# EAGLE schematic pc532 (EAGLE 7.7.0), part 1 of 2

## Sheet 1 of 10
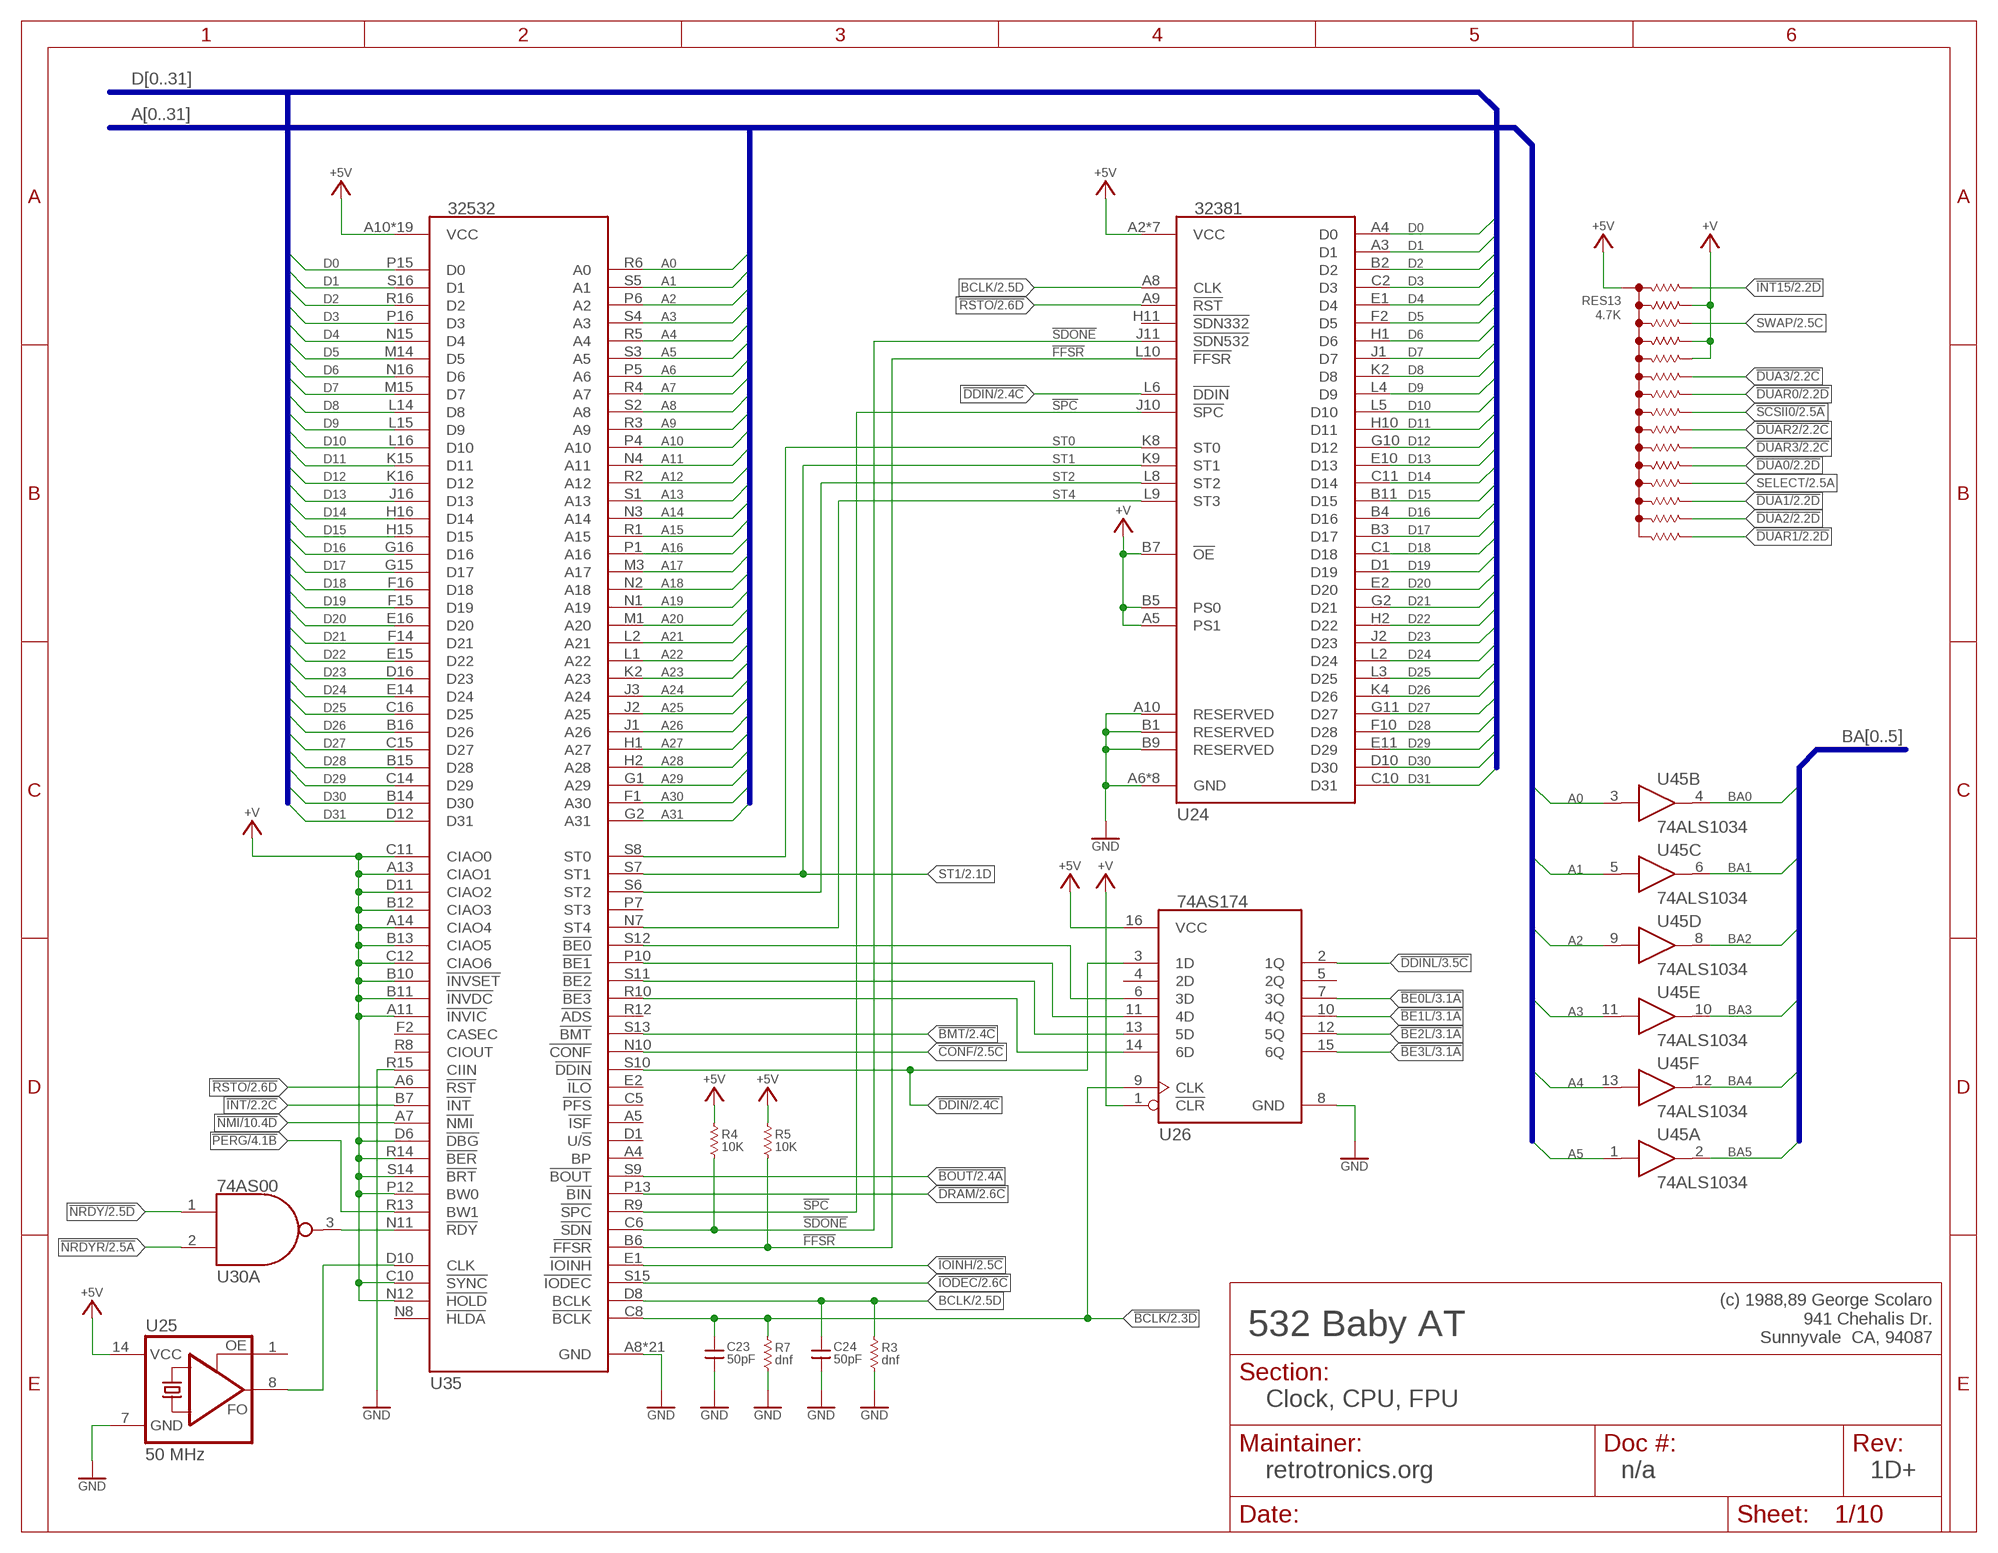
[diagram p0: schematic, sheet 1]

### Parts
C23  50pF  C_US_300M  [C_TH_300MIL]
C24  50pF  C_US_300M  [C_TH_300MIL]
R3  dnf  R_US  [R_204/7]
R4  10K  R_US  [R_204/7]
R5  10K  R_US  [R_204/7]
R7  dnf  R_US  [R_204/7]
RES13  4.7K  RNET_X15  [DIL16]
U24  32381  [PGA68]
U25  50 MHz  XTAL_CAN_HALFSIZEFP  [DIL14]
U26  74AS174  74174  [DIL16]
U30  74AS00  7400  [DIL14]
U35  32532  [PGA175]
U45  74ALS1034  7407D  [DIL14]

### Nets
!BCLK: C23.1 R7.2 U26.9(CLK) U35.C8(!BCLK) ; also sheet 2,3
!BE0: U26.6(3D) U35.S12(!BE0)
!BE0L: U26.7(3Q) ; also sheet 3,10
!BE1: U26.11(4D) U35.P10(!BE1)
!BE1L: U26.10(4Q) ; also sheet 3,10
!BE2: U26.13(5D) U35.S11(!BE2)
!BE2L: U26.12(5Q) ; also sheet 3,10
!BE3: U26.14(6D) U35.R10(!BE3)
!BE3L: U26.15(6Q) ; also sheet 3,10
!BMT: U35.S13(!BMT) ; also sheet 2,3
!BOUT: U35.S9(!BOUT) ; also sheet 2
!CONF: U35.N10(!CONF) ; also sheet 2,3
!DDIN: U24.L6(!DDIN) U26.3(1D) U35.S10(!DDIN) ; also sheet 2,3
!DDINL: U26.2(1Q) ; also sheet 3,4
!DRAM: U35.P13(!BIN) ; also sheet 2,3
!DUA0: RES13.11(R11) ; also sheet 2,7
!DUA1: RES13.13(R13) ; also sheet 2,6
!DUA2: RES13.14(R14) ; also sheet 2,7
!DUA3: RES13.6(R6) ; also sheet 2,6
!DUAR0: RES13.7(R7) ; also sheet 2,7
!DUAR1: RES13.15(R15) ; also sheet 2,6
!DUAR2: RES13.9(R9) ; also sheet 2,7
!DUAR3: RES13.10(R10) ; also sheet 2,6
!FFSR: R5.1 U24.L10(!FFSR) U35.B6(!FFSR)
!INT: U35.B7(!INT) ; also sheet 2
!INT15: RES13.1(R1) ; also sheet 2
!IODEC: U35.S15(!IODEC) ; also sheet 2
!IOINH: U35.E1(!IOINH) ; also sheet 2
!NMI: U35.A7(!NMI) ; also sheet 10
!NRDY: U30.1(A:A) ; also sheet 2
!NRDYR: U30.2(A:B) ; also sheet 2
!PERG: U35.R13(BW1) ; also sheet 4
!RDY: U30.3(A:Y) U35.N11(!RDY)
!RSTO: U24.A9(!RST) U35.A6(!RST) ; also sheet 2,4,5,10
!SCSII0: RES13.8(R8) ; also sheet 2,4
!SDONE: R4.1 U24.J11(!SDN532) U35.C6(!SDN)
!SPC: U24.J10(!SPC) U35.R9(!SPC)
+5V: R4.2 R5.2 RES13.16(C) U24.A2(VCC) U24.B10(VCC) U24.D2(VCC) U24.D11(VCC) U24.K1(VCC) U24.K6(VCC) U24.L7(VCC) U25.14(VCC) U26.16(VCC) U35.A10(VCC) U35.A15(VCC) U35.B2(VCC) U35.B5(VCC) U35.B8(VCC) U35.C3(VCC) U35.C9(VCC) U35.C13(VCC) U35.D15(VCC) U35.G3(VCC) U35.H14(VCC) U35.J15(VCC) U35.K1(VCC) U35.L3(VCC) U35.M16(VCC) U35.N13(VCC) U35.P2(VCC) U35.P9(VCC) U35.R11(VCC) ; also sheet 2,3,4,5,6,7,8,9,10
+V: RES13.2(R2) RES13.4(R4) RES13.5(R5) U24.A5(PS1) U24.B5(PS0) U24.B7(!OE) U26.1(!CLR) U35.A11(!INVIC) U35.A13(CIAO1) U35.A14(CIAO4) U35.B10(!INVSET) U35.B11(!INVDC) U35.B12(CIAO3) U35.B13(CIAO5) U35.C10(!SYNC) U35.C11(CIAO0) U35.C12(CIAO6) U35.D6(!DBG) U35.D11(CIAO2) U35.N12(!HOLD) U35.P12(BW0) U35.R14(!BER) U35.S14(!BRT) ; also sheet 2,3,4
A0: U35.R6(A0) U45.3(B:A) ; also sheet 2
A1: U35.S5(A1) U45.5(C:A) ; also sheet 2
A2: U35.P6(A2) U45.9(D:A) ; also sheet 2,3
A3: U35.S4(A3) U45.11(E:A) ; also sheet 2,3
A4: U35.R5(A4) U45.13(F:A) ; also sheet 2,3
A5: U35.S3(A5) U45.1(A:A) ; also sheet 2,3
A6: U35.P5(A6) ; also sheet 2,3
A7: U35.R4(A7) ; also sheet 2,3
A8: U35.S2(A8) ; also sheet 2,3
A9: U35.R3(A9) ; also sheet 2,3
A10: U35.P4(A10) ; also sheet 2,3
A11: U35.N4(A11) ; also sheet 2,3
A12: U35.R2(A12) ; also sheet 2,3
A13: U35.S1(A13) ; also sheet 2,3
A14: U35.N3(A14) ; also sheet 2,3
A15: U35.R1(A15) ; also sheet 2,3
A16: U35.P1(A16) ; also sheet 2,3
A17: U35.M3(A17) ; also sheet 2,3
A18: U35.N2(A18) ; also sheet 2,3
A19: U35.N1(A19) ; also sheet 2,3
A20: U35.M1(A20) ; also sheet 2,3
A21: U35.L2(A21) ; also sheet 2,3
A22: U35.L1(A22) ; also sheet 2,3
A23: U35.K2(A23) ; also sheet 3
A24: U35.J3(A24) ; also sheet 2,3
A25: U35.J2(A25)
A26: U35.J1(A26)
A27: U35.H1(A27) ; also sheet 2
A28: U35.H2(A28) ; also sheet 2
A29: U35.G1(A29) ; also sheet 2
A30: U35.F1(A30) ; also sheet 2
A31: U35.G2(A31) ; also sheet 2
BA0: U45.4(B:Y) ; also sheet 2,4,5,6,7
BA1: U45.6(C:Y) ; also sheet 2,5,6,7
BA2: U45.8(D:Y) ; also sheet 2,5,6,7
BA3: U45.10(E:Y) ; also sheet 2,6,7
BA4: U45.12(F:Y) ; also sheet 2
BA5: U45.2(A:Y) ; also sheet 2
BCLK: C24.1 R3.2 U24.A8(CLK) U35.D8(BCLK) ; also sheet 2,10
CLK: U25.8(FO) U35.D10(CLK)
D0: U24.A4(D0) U35.P15(D0) ; also sheet 4,8,10
D1: U24.A3(D1) U35.S16(D1) ; also sheet 4,8,10
D2: U24.B2(D2) U35.R16(D2) ; also sheet 4,8,10
D3: U24.C2(D3) U35.P16(D3) ; also sheet 4,8,10
D4: U24.E1(D4) U35.N15(D4) ; also sheet 4,8,10
D5: U24.F2(D5) U35.M14(D5) ; also sheet 4,8,10
D6: U24.H1(D6) U35.N16(D6) ; also sheet 4,8,10
D7: U24.J1(D7) U35.M15(D7) ; also sheet 4,8,10
D8: U24.K2(D8) U35.L14(D8) ; also sheet 8,10
D9: U24.L4(D9) U35.L15(D9) ; also sheet 8,10
D10: U24.L5(D10) U35.L16(D10) ; also sheet 8,10
D11: U24.H10(D11) U35.K15(D11) ; also sheet 8,10
D12: U24.G10(D12) U35.K16(D12) ; also sheet 8,10
D13: U24.E10(D13) U35.J16(D13) ; also sheet 8,10
D14: U24.C11(D14) U35.H16(D14) ; also sheet 8,10
D15: U24.B11(D15) U35.H15(D15) ; also sheet 8,10
D16: U24.B4(D16) U35.G16(D16) ; also sheet 8,10
D17: U24.B3(D17) U35.G15(D17) ; also sheet 8,10
D18: U24.C1(D18) U35.F16(D18) ; also sheet 8,10
D19: U24.D1(D19) U35.F15(D19) ; also sheet 8,10
D20: U24.E2(D20) U35.E16(D20) ; also sheet 8,10
D21: U24.G2(D21) U35.F14(D21) ; also sheet 8,10
D22: U24.H2(D22) U35.E15(D22) ; also sheet 8,10
D23: U24.J2(D23) U35.D16(D23) ; also sheet 8,10
D24: U24.L2(D24) U35.E14(D24) ; also sheet 8,10
D25: U24.L3(D25) U35.C16(D25) ; also sheet 8,10
D26: U24.K4(D26) U35.B16(D26) ; also sheet 8,10
D27: U24.G11(D27) U35.C15(D27) ; also sheet 8,10
D28: U24.F10(D28) U35.B15(D28) ; also sheet 8,10
D29: U24.E11(D29) U35.C14(D29) ; also sheet 8,10
D30: U24.D10(D30) U35.B14(D30) ; also sheet 8,10
D31: U24.C10(D31) U35.D12(D31) ; also sheet 8,10
GND: C23.2 C24.2 R3.1 R7.1 U24.A6(GND) U24.A7(GND) U24.A10(RESERVED) U24.B1(RESERVED) U24.B6(GND) U24.B9(RESERVED) U24.F11(GND) U24.G1(GND) U24.K3(GND) U24.K5(GND) U24.K11(GND) U25.7(GND) U26.8(GND) U35.A8(GND) U35.A12(GND) U35.B9(GND) U35.D4(GND) U35.D5(GND) U35.D9(GND) U35.D13(GND) U35.D14(GND) U35.E3(GND) U35.G14(GND) U35.H3(GND) U35.J14(GND) U35.K3(GND) U35.K14(GND) U35.M2(GND) U35.N6(GND) U35.N9(GND) U35.N14(GND) U35.P3(GND) U35.P8(GND) U35.P11(GND) U35.R15(CIIN) ; also sheet 2,3,4,5,6,7,8,9,10
SELECT: RES13.12(R12) ; also sheet 2
ST0: U24.K8(ST0) U35.S8(ST0)
ST1: U24.K9(ST1) U35.S7(ST1) ; also sheet 2
ST2: U24.L8(ST2) U35.S6(ST2)
ST4: U24.L9(ST3) U35.N7(ST4)
SWAP: RES13.3(R3) ; also sheet 2
Unconnected: U24.H11(!SDN332) U25.1(OE) U26.4(2D) U26.5(2Q) U35.A4(BP) U35.A5(!ISF) U35.C5(!PFS) U35.D1(U/!S) U35.E2(!ILO) U35.F2(CASEC) U35.N8(!HLDA) U35.P7(ST3) U35.R8(CIOUT) U35.R12(!ADS)

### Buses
D[0..31]
A[0..31]
BA[0..5]

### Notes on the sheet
- (c) 1988,89 George Scolaro
  941 Chehalis Dr.
  Sunnyvale  CA, 94087
- 532 Baby AT
- Clock, CPU, FPU
- retrotronics.org | n/a | 1D+

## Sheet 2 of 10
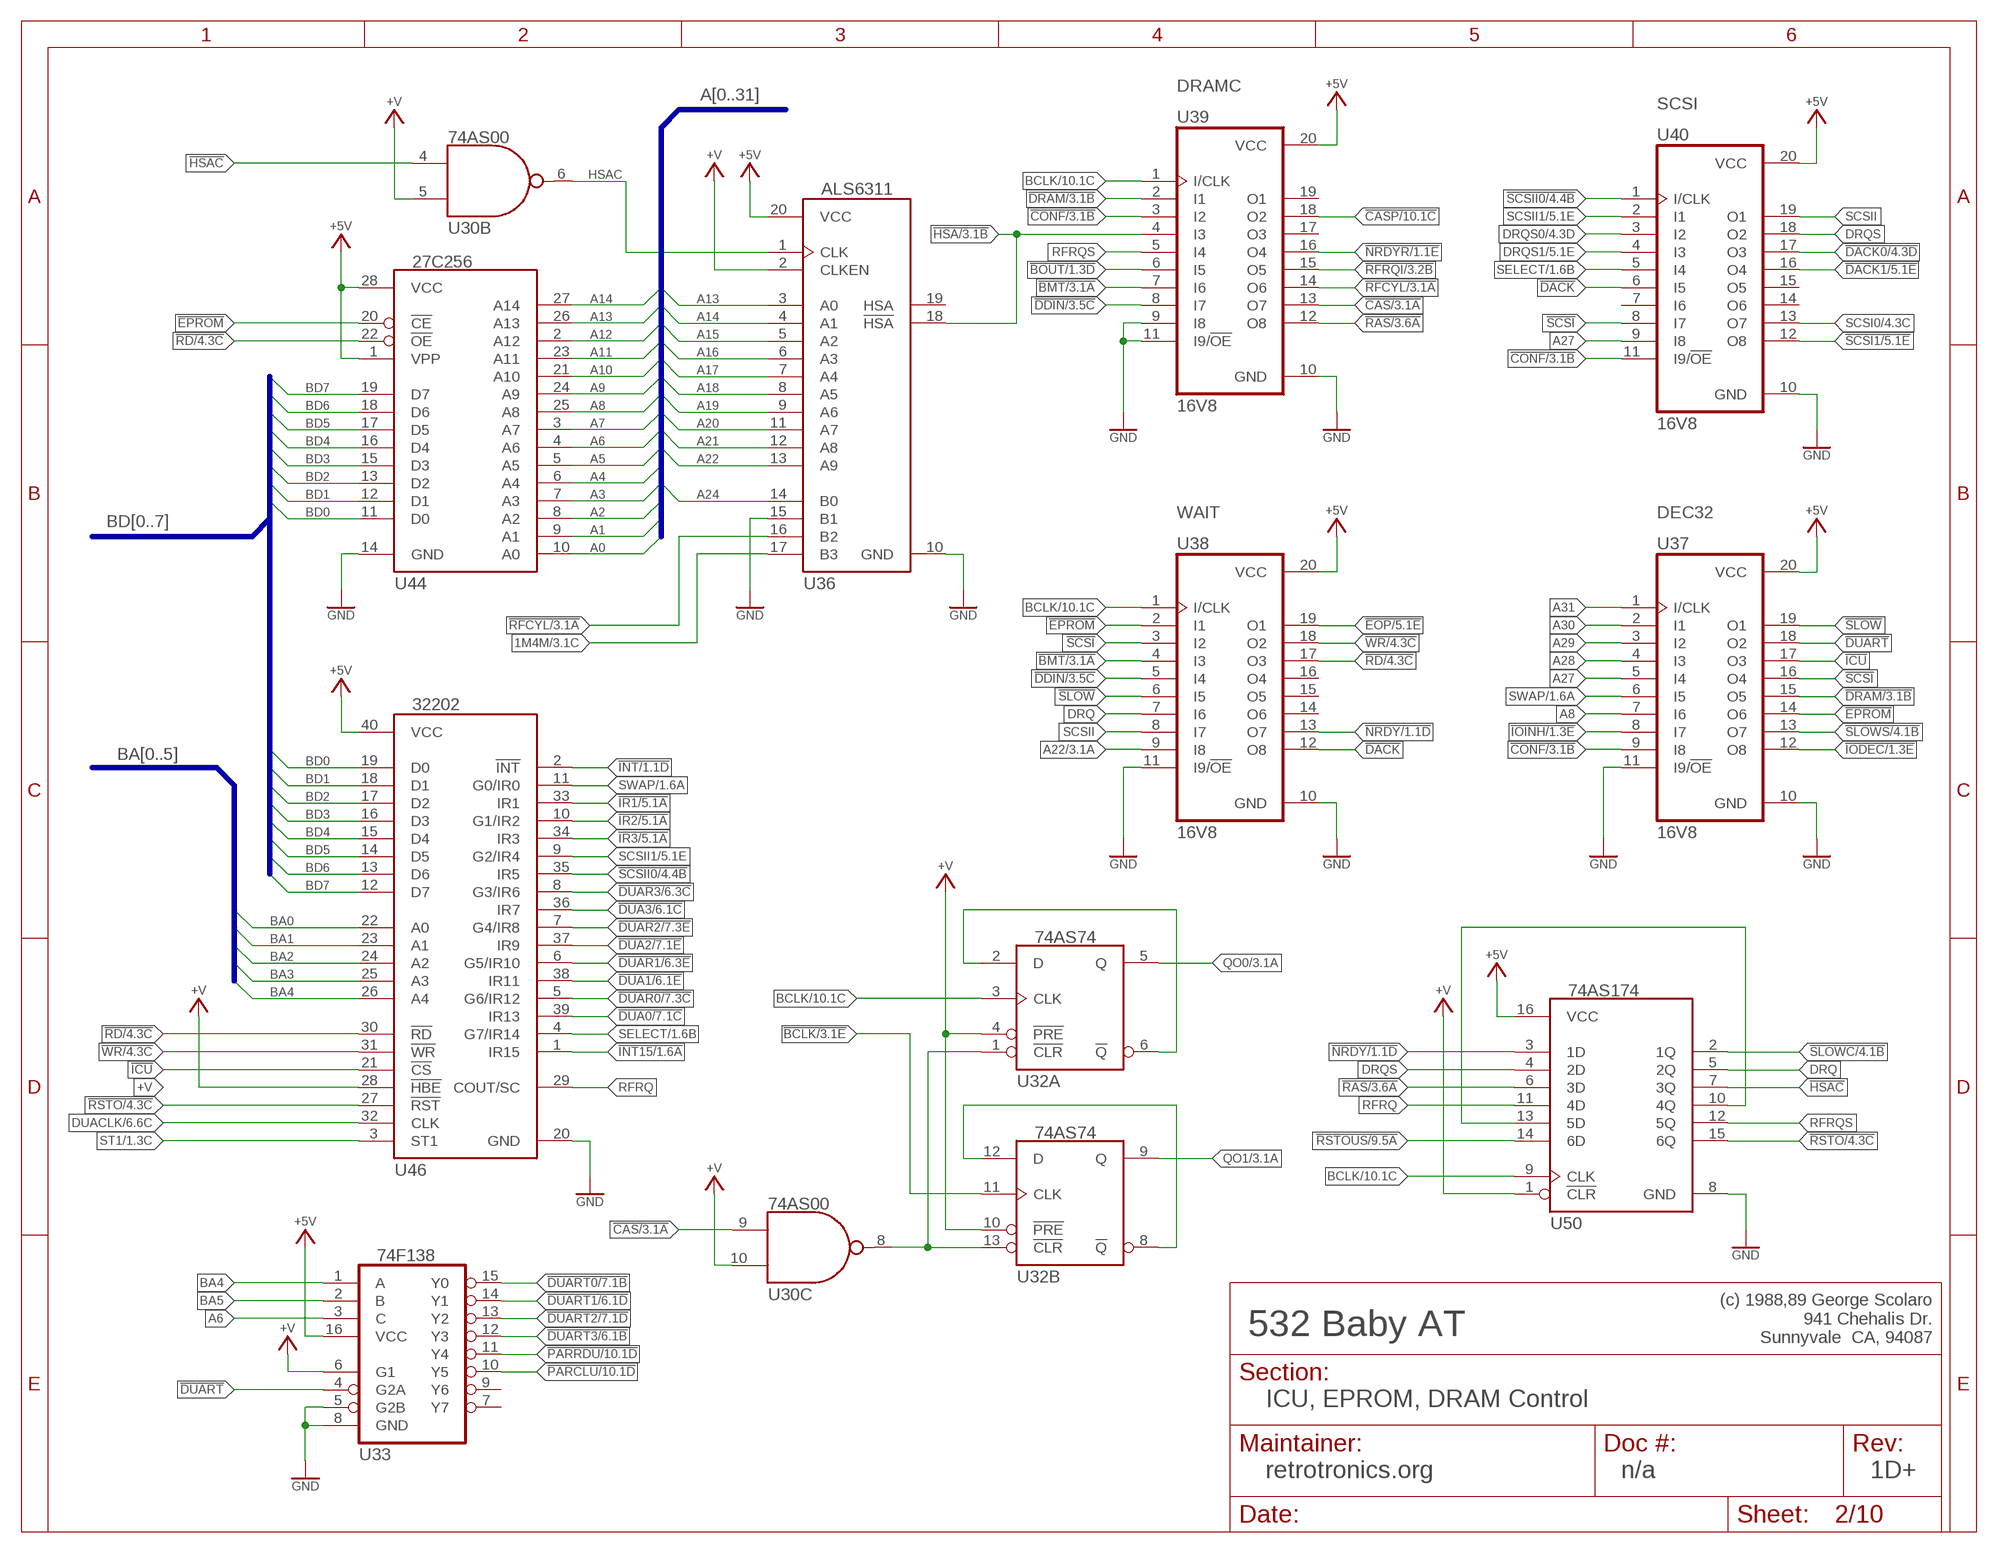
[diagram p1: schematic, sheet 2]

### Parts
U32  74AS74  7474  [DIL14]
U33  74F138  74138  [DIL16]
U36  ALS6311  746311  [DIL20]
U37  16V8  16V8_RND  [DIL20_ROUND]
U38  16V8  16V8_RND  [DIL20_ROUND]
U39  16V8  16V8_RND  [DIL20_ROUND]
U40  16V8  16V8_RND  [DIL20_ROUND]
U44  27C256  [DIL28W]
U46  32202  [DIL40]
U50  74AS174  74174  [DIL16]

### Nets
1M4M: U36.17(B3) ; also sheet 3
!BCLK: U32.11(B:CLK) ; also sheet 1,3
!BCLK_CLR: U30.8(C:Y) U32.1(A:!CLR) U32.13(B:!CLR)
!BMT: U38.4(I3) U39.7(I6) ; also sheet 1,3
!BOUT: U39.6(I5) ; also sheet 1
!CAS: U30.9(C:A) U39.13(O7) ; also sheet 3
!CASP: U39.18(O2) ; also sheet 10
!CONF: U37.9(I8) U39.3(I2) U40.11(I9/!OE) ; also sheet 1,3
!DACK: U38.12(O8) U40.6(I5)
!DACK0: U40.17(O3) ; also sheet 4
!DACK1: U40.16(O4) ; also sheet 5
!DDIN: U38.5(I4) U39.8(I7) ; also sheet 1,3
!DRAM: U37.15(O5) U39.2(I1) ; also sheet 1,3
!DUA0: U46.39(IR13) ; also sheet 1,7
!DUA1: U46.38(IR11) ; also sheet 1,6
!DUA2: U46.37(IR9) ; also sheet 1,7
!DUA3: U46.36(IR7) ; also sheet 1,6
!DUAR0: U46.5(G6/IR12) ; also sheet 1,7
!DUAR1: U46.6(G5/IR10) ; also sheet 1,6
!DUAR2: U46.7(G4/IR8) ; also sheet 1,7
!DUAR3: U46.8(G3/IR6) ; also sheet 1,6
!DUART: U33.4(G2A) U37.18(O2)
!DUART0: U33.15(Y0) ; also sheet 7
!DUART1: U33.14(Y1) ; also sheet 6
!DUART2: U33.13(Y2) ; also sheet 7
!DUART3: U33.12(Y3) ; also sheet 6
!EOP: U38.19(O1) ; also sheet 5
!EPROM: U37.14(O6) U38.2(I1) U44.20(!CE)
!HSA: U36.18(!HSA) U39.4(I3) ; also sheet 3
!HSAC: U30.4(B:A) U50.7(3Q)
!ICU: U37.17(O3) U46.21(!CS)
!INT: U46.2(!INT) ; also sheet 1
!INT15: U46.1(IR15) ; also sheet 1
!IODEC: U37.12(O8) ; also sheet 1
!IOINH: U37.8(I7) ; also sheet 1
!IR1: U46.33(IR1) ; also sheet 5
!IR2: U46.10(G1/IR2) ; also sheet 5
!IR3: U46.34(IR3) ; also sheet 5
!NRDY: U38.13(O7) U50.3(1D) ; also sheet 1
!NRDYR: U39.16(O4) ; also sheet 1
!PARCLU: U33.10(Y5) ; also sheet 10
!PARRDU: U33.11(Y4) ; also sheet 10
!RAS: U39.12(O8) U50.6(3D) ; also sheet 3
!RD: U38.17(O3) U44.22(!OE) U46.30(!RD) ; also sheet 4,5,6,7,10
!RFCYL: U36.16(B2) U39.14(O6) ; also sheet 3
!RFRQI: U39.15(O5) ; also sheet 3
!RSTO: U46.27(!RST) U50.15(6Q) ; also sheet 1,4,5,10
!RSTOUS: U50.14(6D) ; also sheet 9
!SCSI: U37.16(O4) U38.3(I2) U40.8(I7)
!SCSI1: U40.12(O8) ; also sheet 5
!SCSII0: U40.1(I/CLK) U46.35(IR5) ; also sheet 1,4
!SLOW: U37.19(O1) U38.6(I5)
!SLOWC: U50.2(1Q) ; also sheet 4
!SLOWS: U37.13(O7) ; also sheet 4
!WR: U38.18(O2) U46.31(!WR) ; also sheet 4,5,6,7
+5V: U33.16(VCC) U36.20(VCC) U37.20(VCC) U38.20(VCC) U39.20(VCC) U40.20(VCC) U44.1(VPP) U44.28(VCC) U46.40(VCC) U50.16(VCC) ; also sheet 1,3,4,5,6,7,8,9,10
+V: U30.5(B:B) U30.10(C:B) U32.4(A:!PRE) U32.10(B:!PRE) U33.6(G1) U36.2(CLKEN) U46.28(!HBE) U50.1(!CLR) ; also sheet 1,3,4
A0: U44.10(A0) ; also sheet 1
A1: U44.9(A1) ; also sheet 1
A2: U44.8(A2) ; also sheet 1,3
A3: U44.7(A3) ; also sheet 1,3
A4: U44.6(A4) ; also sheet 1,3
A5: U44.5(A5) ; also sheet 1,3
A6: U33.3(C) U44.4(A6) ; also sheet 1,3
A7: U44.3(A7) ; also sheet 1,3
A8: U37.7(I6) U44.25(A8) ; also sheet 1,3
A9: U44.24(A9) ; also sheet 1,3
A10: U44.21(A10) ; also sheet 1,3
A11: U44.23(A11) ; also sheet 1,3
A12: U44.2(A12) ; also sheet 1,3
A13: U36.3(A0) U44.26(A13) ; also sheet 1,3
A14: U36.4(A1) U44.27(A14) ; also sheet 1,3
A15: U36.5(A2) ; also sheet 1,3
A16: U36.6(A3) ; also sheet 1,3
A17: U36.7(A4) ; also sheet 1,3
A18: U36.8(A5) ; also sheet 1,3
A19: U36.9(A6) ; also sheet 1,3
A20: U36.11(A7) ; also sheet 1,3
A21: U36.12(A8) ; also sheet 1,3
A22: U36.13(A9) U38.9(I8) ; also sheet 1,3
A24: U36.14(B0) ; also sheet 1,3
A27: U37.5(I4) U40.9(I8) ; also sheet 1
A28: U37.4(I3) ; also sheet 1
A29: U37.3(I2) ; also sheet 1
A30: U37.2(I1) ; also sheet 1
A31: U37.1(I/CLK) ; also sheet 1
BA0: U46.22(A0) ; also sheet 1,4,5,6,7
BA1: U46.23(A1) ; also sheet 1,5,6,7
BA2: U46.24(A2) ; also sheet 1,5,6,7
BA3: U46.25(A3) ; also sheet 1,6,7
BA4: U33.1(A) U46.26(A4) ; also sheet 1
BA5: U33.2(B) ; also sheet 1
BCLK: U32.3(A:CLK) U38.1(I/CLK) U39.1(I/CLK) U50.9(CLK) ; also sheet 1,10
BD0: U44.11(D0) U46.19(D0) ; also sheet 4,5,6,7,10
BD1: U44.12(D1) U46.18(D1) ; also sheet 4,5,6,7,10
BD2: U44.13(D2) U46.17(D2) ; also sheet 4,5,6,7,10
BD3: U44.15(D3) U46.16(D3) ; also sheet 4,5,6,7,10
BD4: U44.16(D4) U46.15(D4) ; also sheet 4,5,6,7,10
BD5: U44.17(D5) U46.14(D5) ; also sheet 4,5,6,7
BD6: U44.18(D6) U46.13(D6) ; also sheet 4,5,6,7
BD7: U44.19(D7) U46.12(D7) ; also sheet 4,5,6,7
DRQ: U38.7(I6) U50.5(2Q)
DRQS: U40.18(O2) U50.4(2D)
DRQS0: U40.3(I2) ; also sheet 4
DRQS1: U40.4(I3) ; also sheet 5
DUACLK: U46.32(CLK) ; also sheet 6,7
FB1: U50.10(4Q) U50.13(5D)
GND: U33.5(G2B) U33.8(GND) U36.10(GND) U36.15(B1) U37.10(GND) U37.11(I9/!OE) U38.10(GND) U38.11(I9/!OE) U39.9(I8) U39.10(GND) U39.11(I9/!OE) U40.10(GND) U44.14(GND) U46.20(GND) U50.8(GND) ; also sheet 1,3,4,5,6,7,8,9,10
HSAC: U30.6(B:Y) U36.1(CLK)
QF0: U32.2(A:D) U32.6(A:!Q)
QF1: U32.8(B:!Q) U32.12(B:D)
QO0: U32.5(A:Q) ; also sheet 3
QO1: U32.9(B:Q) ; also sheet 3
RFRQ: U46.29(COUT/SC) U50.11(4D)
RFRQS: U39.5(I4) U50.12(5Q)
SCSI0: U40.13(O7) ; also sheet 4
SCSII: U38.8(I7) U40.19(O1)
SCSII1: U40.2(I1) U46.9(G2/IR4) ; also sheet 5
SELECT: U40.5(I4) U46.4(G7/IR14) ; also sheet 1
ST1: U46.3(ST1) ; also sheet 1
SWAP: U37.6(I5) U46.11(G0/IR0) ; also sheet 1
Unconnected: U33.7(Y7) U33.9(Y6) U36.19(HSA) U38.14(O6) U38.15(O5) U38.16(O4) U39.17(O3) U39.19(O1) U40.7(I6) U40.14(O6) U40.15(O5)

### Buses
BD[0..7]
A[0..31]
BA[0..5]

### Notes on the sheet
- DRAMC
- SCSI
- WAIT | DEC32
- (c) 1988,89 George Scolaro
  941 Chehalis Dr.
  Sunnyvale  CA, 94087
- 532 Baby AT
- ICU, EPROM, DRAM Control
- retrotronics.org | n/a | 1D+

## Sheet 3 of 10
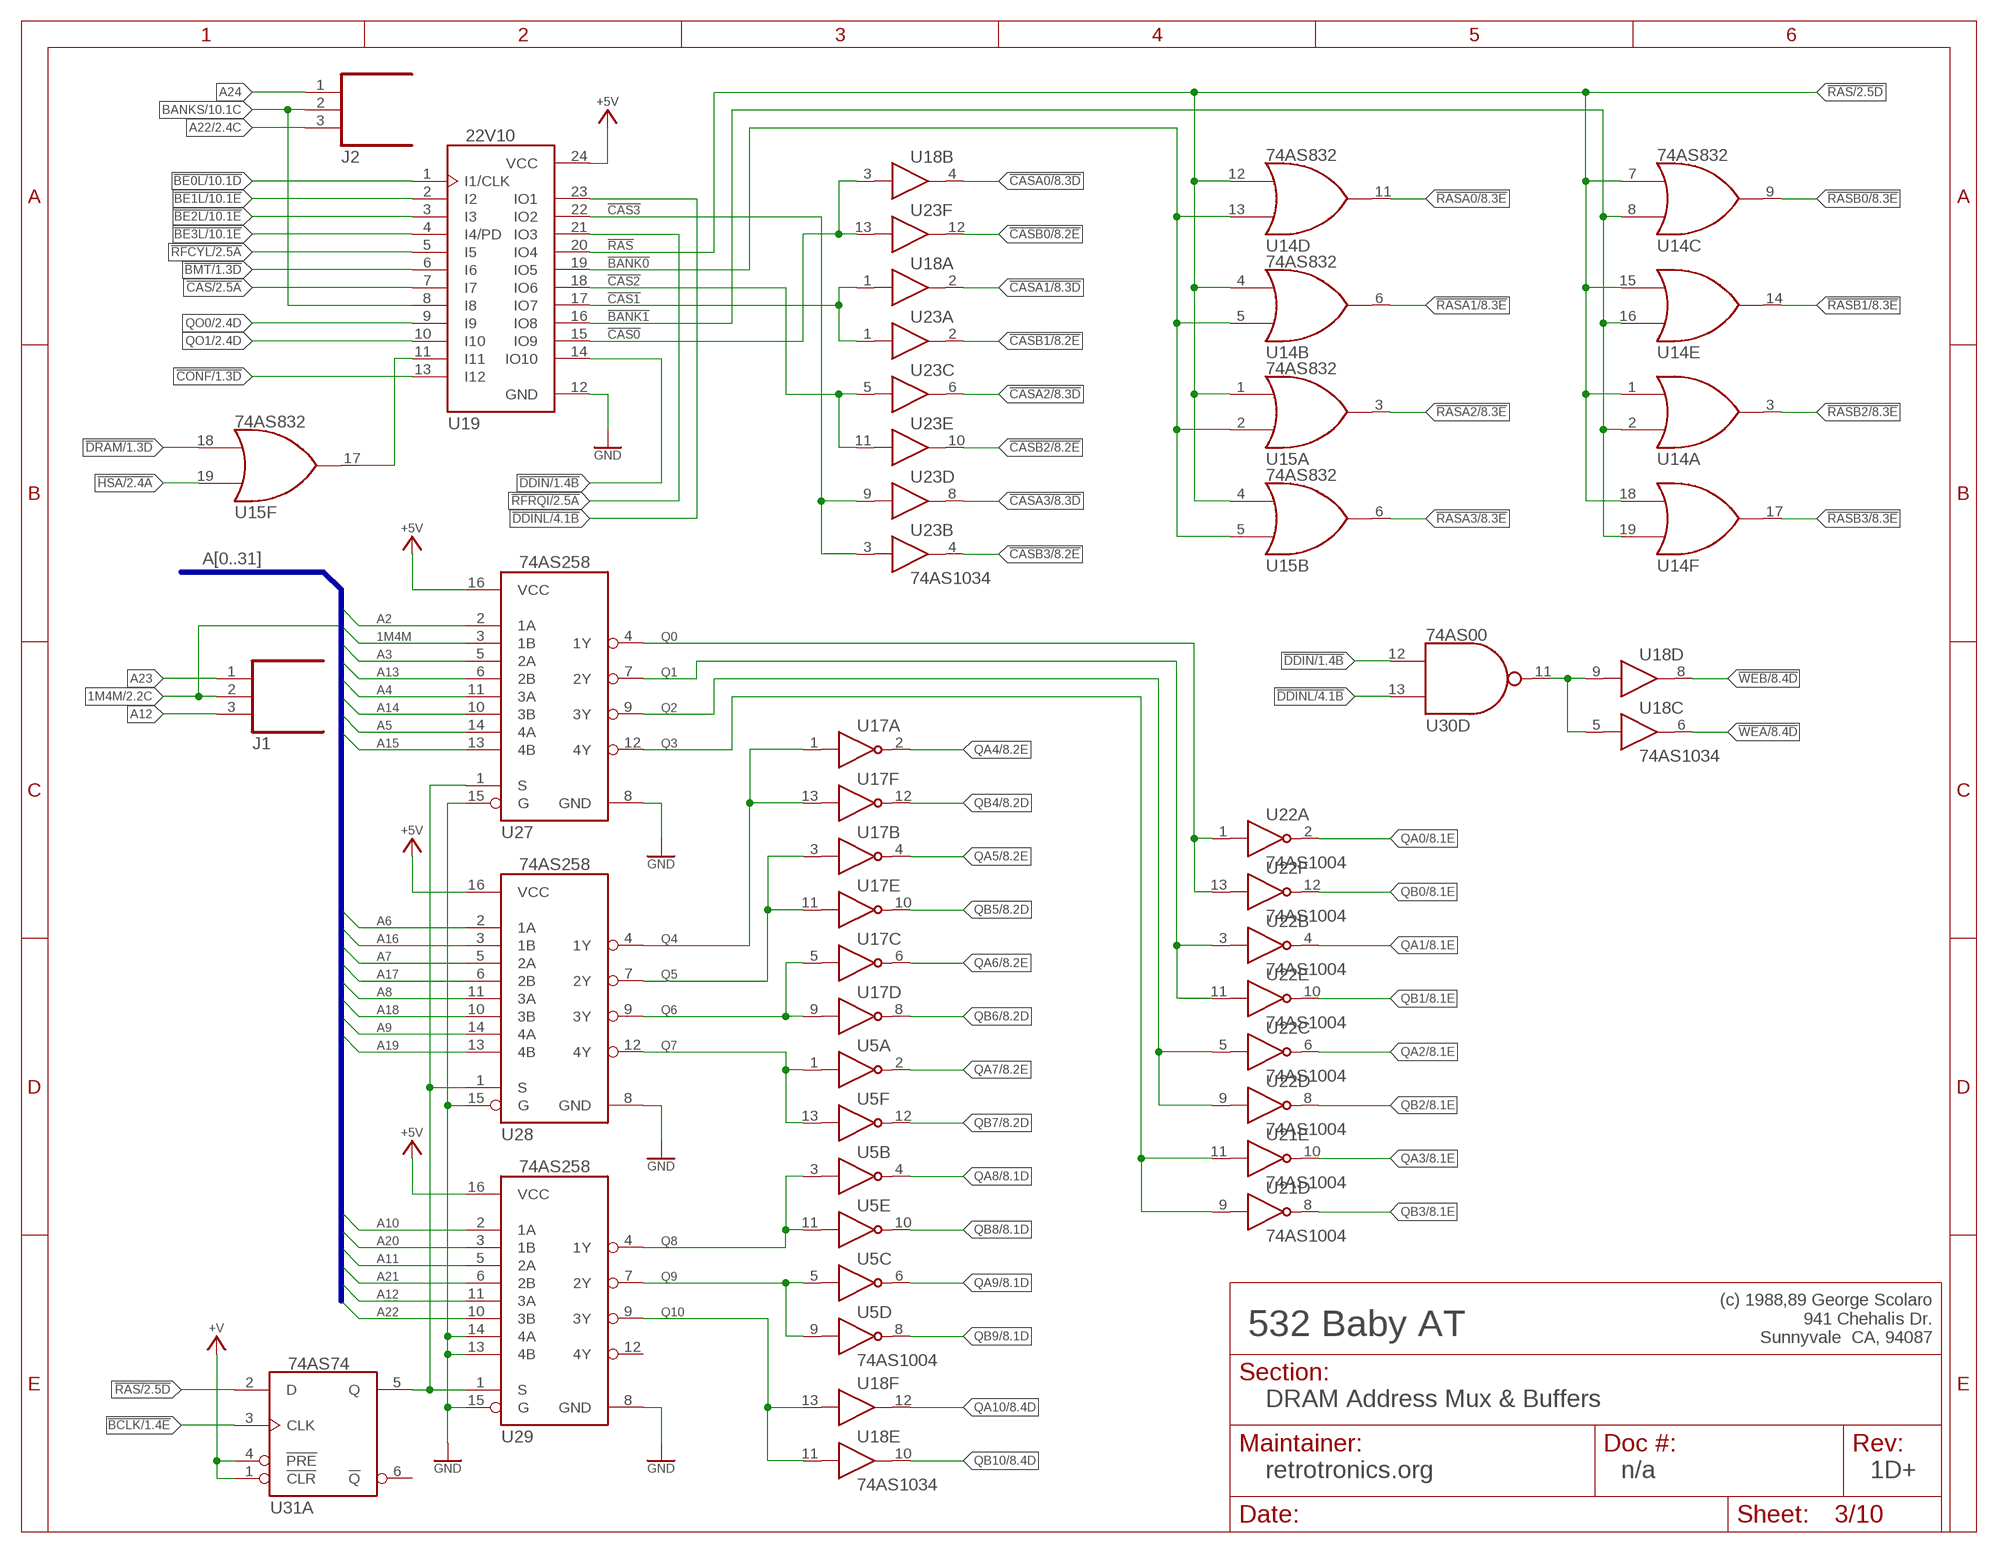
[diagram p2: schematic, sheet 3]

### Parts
J1  HDR_1X3N  [HDR_1X3]
J2  HDR_1X3N  [HDR_1X3]
U5  74AS1004  7404  [DIL14]
U14  74AS832  74832  [DIL20]
U15  74AS832  74832  [DIL20]
U17  74AS1004  7404  [DIL14]
U18  74AS1034  7407D  [DIL14]
U19  22V10  22V10P  [DIL24]
U21  74AS1004  7404  [DIL14]
U22  74AS1004  7404  [DIL14]
U23  74AS1034  7407D  [DIL14]
U27  74AS258  74258  [DIL16]
U28  74AS258  74258  [DIL16]
U29  74AS258  74258  [DIL16]
U31  74AS74  7474  [DIL14]

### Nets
1M4M: J1.2 U27.3(1B) ; also sheet 2
!BANK0: U14.5(B:B) U14.13(D:B) U15.2(A:B) U15.5(B:B) U19.19(IO5)
!BANK1: U14.2(A:B) U14.8(C:B) U14.16(E:B) U14.19(F:B) U19.16(IO8)
!BCLK: U31.3(A:CLK) ; also sheet 1,2
!BE0L: U19.1(I1/CLK) ; also sheet 1,10
!BE1L: U19.2(I2) ; also sheet 1,10
!BE2L: U19.3(I3) ; also sheet 1,10
!BE3L: U19.4(I4/PD) ; also sheet 1,10
!BMT: U19.6(I6) ; also sheet 1,2
!CAS: U19.7(I7) ; also sheet 2
!CAS0: U18.3(B:A) U19.15(IO9) U23.13(F:A)
!CAS1: U18.1(A:A) U19.17(IO7) U23.1(A:A)
!CAS2: U19.18(IO6) U23.5(C:A) U23.11(E:A)
!CAS3: U19.22(IO2) U23.3(B:A) U23.9(D:A)
!CASA0: U18.4(B:Y) ; also sheet 8
!CASA1: U18.2(A:Y) ; also sheet 8
!CASA2: U23.6(C:Y) ; also sheet 8
!CASA3: U23.8(D:Y) ; also sheet 8
!CASB0: U23.12(F:Y) ; also sheet 8
!CASB1: U23.2(A:Y) ; also sheet 8
!CASB2: U23.10(E:Y) ; also sheet 8
!CASB3: U23.4(B:Y) ; also sheet 8
!CONF: U19.13(I12) ; also sheet 1,2
!DDIN: U19.14(IO10) U30.12(D:A) ; also sheet 1,2
!DDINL: U19.23(IO1) U30.13(D:B) ; also sheet 1,4
!DRAM: U15.18(F:A) ; also sheet 1,2
!HSA: U15.19(F:B) ; also sheet 2
!HSADR: U15.17(F:Y) U19.11(I11)
!RAS: U14.1(A:A) U14.4(B:A) U14.7(C:A) U14.12(D:A) U14.15(E:A) U14.18(F:A) U15.1(A:A) U15.4(B:A) U19.20(IO4) U31.2(A:D) ; also sheet 2
!RASA0: U14.11(D:Y) ; also sheet 8
!RASA1: U14.6(B:Y) ; also sheet 8
!RASA2: U15.3(A:Y) ; also sheet 8
!RASA3: U15.6(B:Y) ; also sheet 8
!RASB0: U14.9(C:Y) ; also sheet 8
!RASB1: U14.14(E:Y) ; also sheet 8
!RASB2: U14.3(A:Y) ; also sheet 8
!RASB3: U14.17(F:Y) ; also sheet 8
!RFCYL: U19.5(I5) ; also sheet 2
!RFRQI: U19.21(IO3) ; also sheet 2
!WEA: U18.6(C:Y) ; also sheet 8
!WEAB: U18.5(C:A) U18.9(D:A) U30.11(D:Y)
!WEB: U18.8(D:Y) ; also sheet 8
+5V: U19.24(VCC) U27.16(VCC) U28.16(VCC) U29.16(VCC) ; also sheet 1,2,4,5,6,7,8,9,10
+V: U31.1(A:!CLR) U31.4(A:!PRE) ; also sheet 1,2,4
A2: U27.2(1A) ; also sheet 1,2
A3: U27.5(2A) ; also sheet 1,2
A4: U27.11(3A) ; also sheet 1,2
A5: U27.14(4A) ; also sheet 1,2
A6: U28.2(1A) ; also sheet 1,2
A7: U28.5(2A) ; also sheet 1,2
A8: U28.11(3A) ; also sheet 1,2
A9: U28.14(4A) ; also sheet 1,2
A10: U29.2(1A) ; also sheet 1,2
A11: U29.5(2A) ; also sheet 1,2
A12: J1.3 U29.11(3A) ; also sheet 1,2
A13: U27.6(2B) ; also sheet 1,2
A14: U27.10(3B) ; also sheet 1,2
A15: U27.13(4B) ; also sheet 1,2
A16: U28.3(1B) ; also sheet 1,2
A17: U28.6(2B) ; also sheet 1,2
A18: U28.10(3B) ; also sheet 1,2
A19: U28.13(4B) ; also sheet 1,2
A20: U29.3(1B) ; also sheet 1,2
A21: U29.6(2B) ; also sheet 1,2
A22: J2.3 U29.10(3B) ; also sheet 1,2
A23: J1.1 ; also sheet 1
A24: J2.1 ; also sheet 1,2
ASEL: U27.1(S) U28.1(S) U29.1(S) U31.5(A:Q)
BANKS: J2.2 U19.8(I8) ; also sheet 10
GND: U19.12(GND) U27.8(GND) U27.15(G) U28.8(GND) U28.15(G) U29.8(GND) U29.13(4B) U29.14(4A) U29.15(G) ; also sheet 1,2,4,5,6,7,8,9,10
Q0: U22.1(A:A) U22.13(F:A) U27.4(1Y)
Q1: U22.3(B:A) U22.11(E:A) U27.7(2Y)
Q2: U22.5(C:A) U22.9(D:A) U27.9(3Y)
Q3: U21.9(D:A) U21.11(E:A) U27.12(4Y)
Q4: U17.1(A:A) U17.13(F:A) U28.4(1Y)
Q5: U17.3(B:A) U17.11(E:A) U28.7(2Y)
Q6: U17.5(C:A) U17.9(D:A) U28.9(3Y)
Q7: U5.1(A:A) U5.13(F:A) U28.12(4Y)
Q8: U5.3(B:A) U5.11(E:A) U29.4(1Y)
Q9: U5.5(C:A) U5.9(D:A) U29.7(2Y)
Q10: U18.11(E:A) U18.13(F:A) U29.9(3Y)
QA0: U22.2(A:Y) ; also sheet 8
QA1: U22.4(B:Y) ; also sheet 8
QA2: U22.6(C:Y) ; also sheet 8
QA3: U21.10(E:Y) ; also sheet 8
QA4: U17.2(A:Y) ; also sheet 8
QA5: U17.4(B:Y) ; also sheet 8
QA6: U17.6(C:Y) ; also sheet 8
QA7: U5.2(A:Y) ; also sheet 8
QA8: U5.4(B:Y) ; also sheet 8
QA9: U5.6(C:Y) ; also sheet 8
QA10: U18.12(F:Y) ; also sheet 8
QB0: U22.12(F:Y) ; also sheet 8
QB1: U22.10(E:Y) ; also sheet 8
QB2: U22.8(D:Y) ; also sheet 8
QB3: U21.8(D:Y) ; also sheet 8
QB4: U17.12(F:Y) ; also sheet 8
QB5: U17.10(E:Y) ; also sheet 8
QB6: U17.8(D:Y) ; also sheet 8
QB7: U5.12(F:Y) ; also sheet 8
QB8: U5.10(E:Y) ; also sheet 8
QB9: U5.8(D:Y) ; also sheet 8
QB10: U18.10(E:Y) ; also sheet 8
QO0: U19.9(I9) ; also sheet 2
QO1: U19.10(I10) ; also sheet 2
Unconnected: U29.12(4Y) U31.6(A:!Q)

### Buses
A[0..31]

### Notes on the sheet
- (c) 1988,89 George Scolaro
  941 Chehalis Dr.
  Sunnyvale  CA, 94087
- 532 Baby AT
- DRAM Address Mux & Buffers
- retrotronics.org | n/a | 1D+

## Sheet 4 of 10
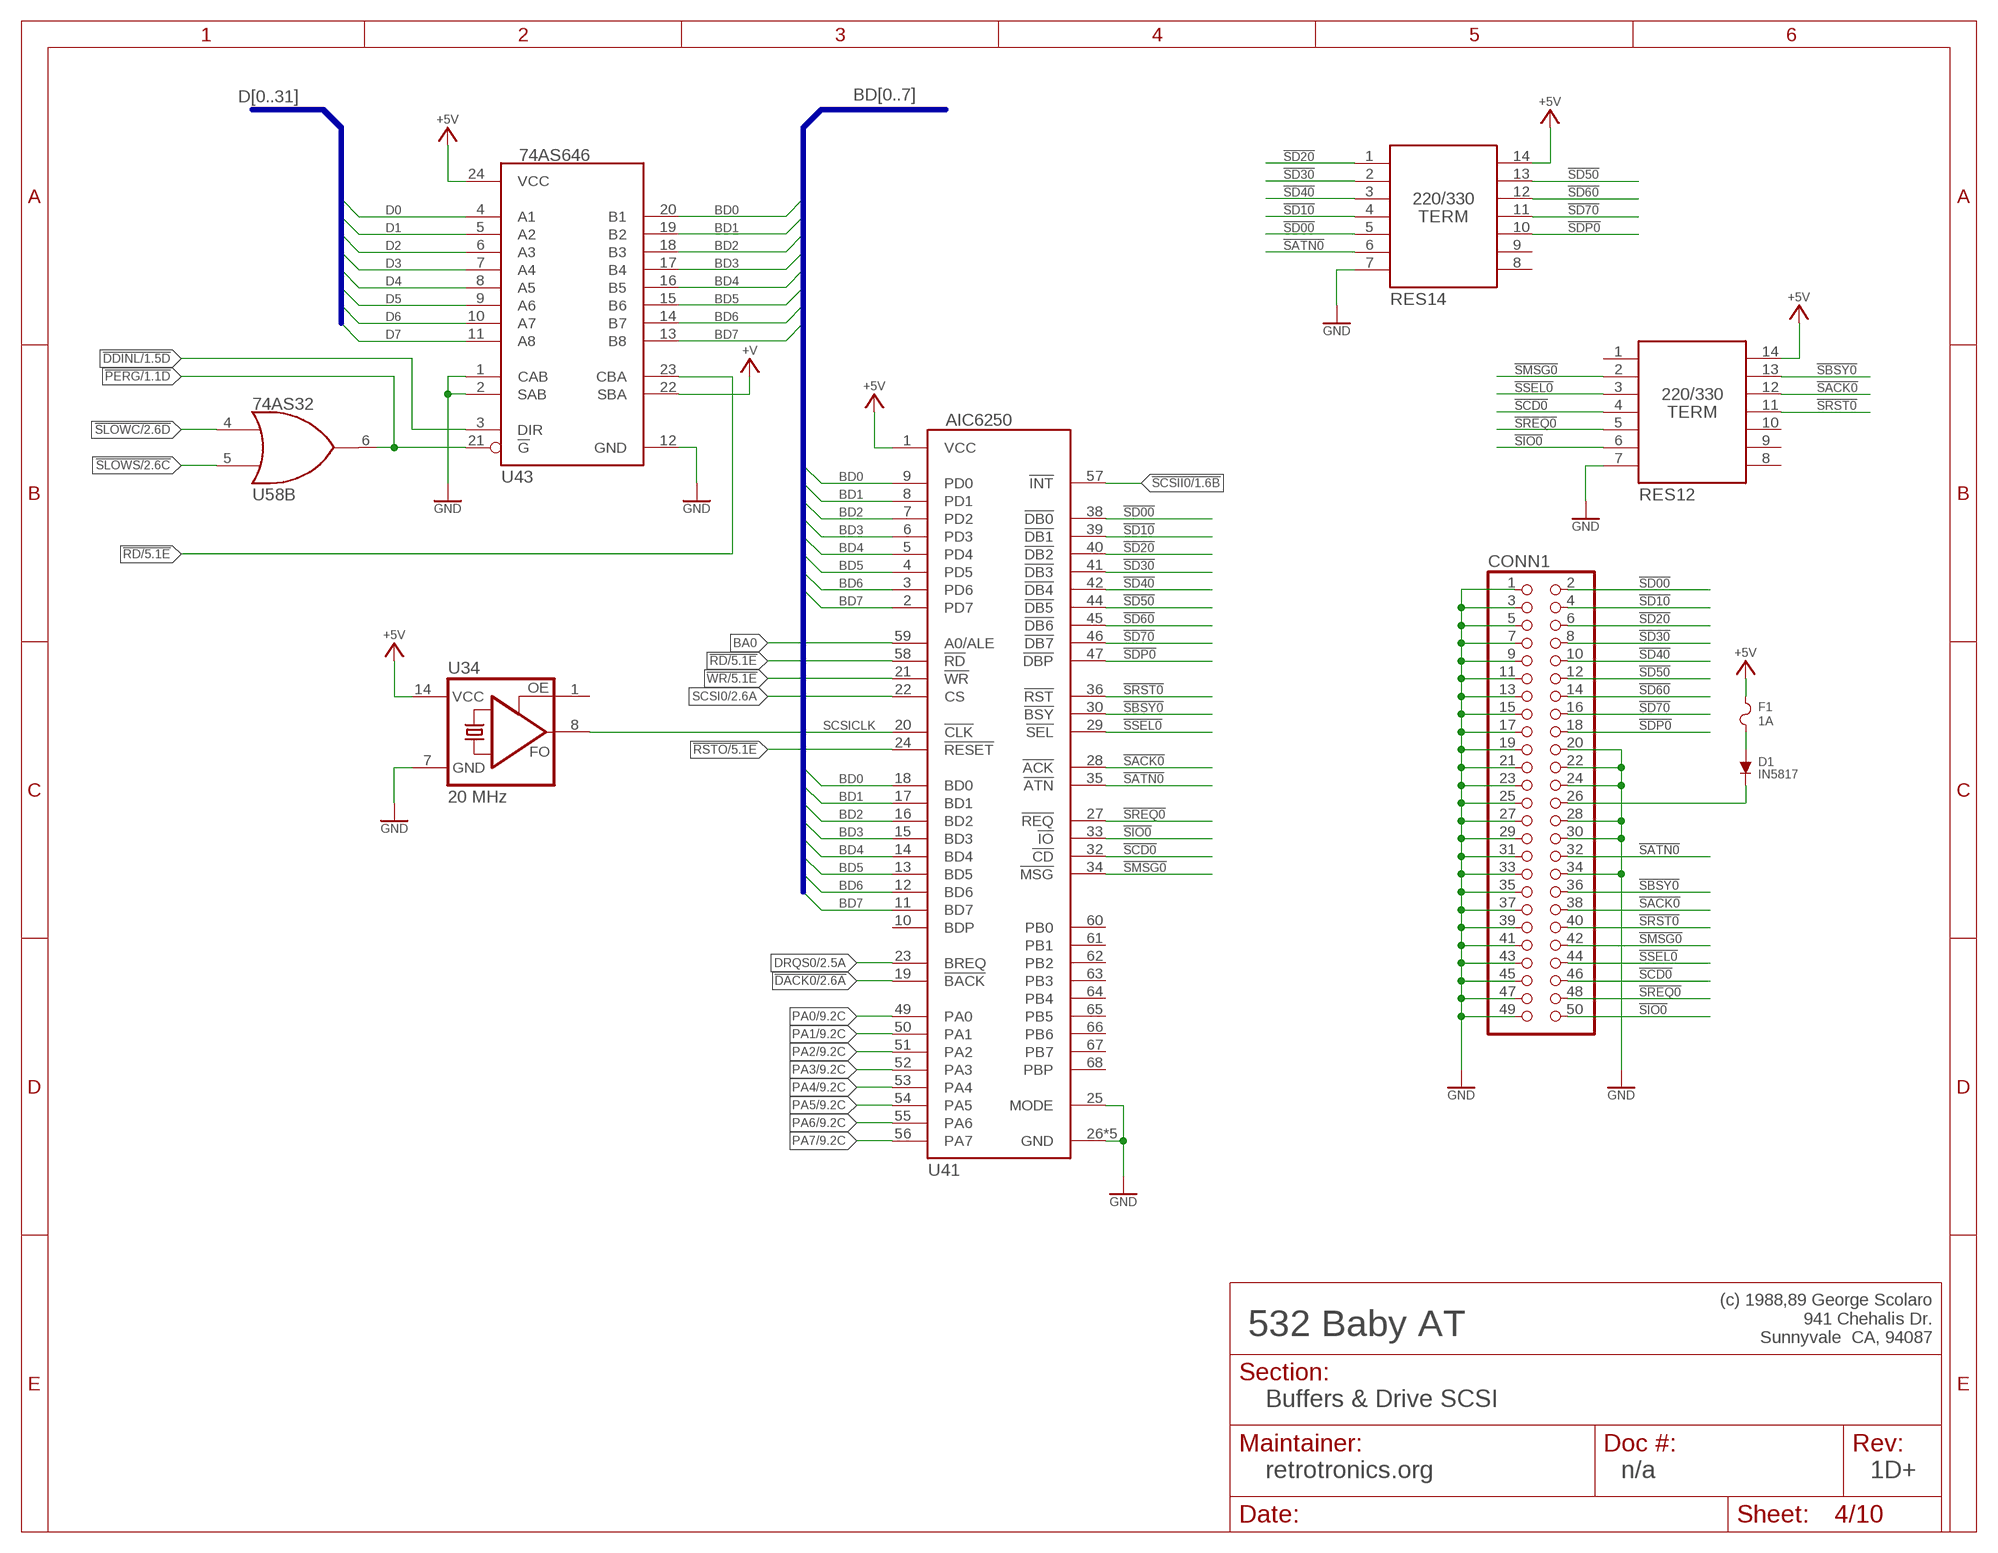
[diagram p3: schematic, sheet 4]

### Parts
CONN1  HDR_2X25  [HDR_2X25]
D1  IN5817  D  [DO35]
F1  1A  FUSE  [FUSE]
RES12  220/330  SCSITERM  [DIL14]
RES14  220/330  SCSITERM  [DIL14]
U34  20 MHz  XTAL_CAN_HALFSIZEFP  [DIL14]
U41  AIC6250  [PLCC68]
U43  74AS646  74646  [DIL24]
U58  74AS32  7432  [DIL14]

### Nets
!DACK0: U41.19(!BACK) ; also sheet 2
!DDINL: U43.3(DIR) ; also sheet 1,3
!PERG: U43.21(!G) U58.6(B:Y) ; also sheet 1
!RD: U41.58(!RD) U43.23(CBA) ; also sheet 2,5,6,7,10
!RSTO: U41.24(!RESET) ; also sheet 1,2,5,10
!SACK0: CONN1.38 RES12.12 U41.28(!ACK)
!SATN0: CONN1.32 RES14.6 U41.35(!ATN)
!SBSY0: CONN1.36 RES12.13 U41.30(!BSY)
!SCD0: CONN1.46 RES12.4 U41.32(!CD)
!SCSII0: U41.57(!INT) ; also sheet 1,2
!SD00: CONN1.2 RES14.5 U41.38(!DB0)
!SD10: CONN1.4 RES14.4 U41.39(!DB1)
!SD20: CONN1.6 RES14.1 U41.40(!DB2)
!SD30: CONN1.8 RES14.2 U41.41(!DB3)
!SD40: CONN1.10 RES14.3 U41.42(!DB4)
!SD50: CONN1.12 RES14.13 U41.44(!DB5)
!SD60: CONN1.14 RES14.12 U41.45(!DB6)
!SD70: CONN1.16 RES14.11 U41.46(!DB7)
!SDP0: CONN1.18 RES14.10 U41.47(!DBP)
!SIO0: CONN1.50 RES12.6 U41.33(!IO)
!SLOWC: U58.4(B:A) ; also sheet 2
!SLOWS: U58.5(B:B) ; also sheet 2
!SMSG0: CONN1.42 RES12.2 U41.34(!MSG)
!SREQ0: CONN1.48 RES12.5 U41.27(!REQ)
!SRST0: CONN1.40 RES12.11 U41.36(!RST)
!SSEL0: CONN1.44 RES12.3 U41.29(!SEL)
!WR: U41.21(!WR) ; also sheet 2,5,6,7
+5V: F1.2 RES12.14 RES14.14 U34.14(VCC) U41.1(VCC) U43.24(VCC) ; also sheet 1,2,3,5,6,7,8,9,10
+V: U43.22(SBA) ; also sheet 1,2,3
_STERM0: D1.A F1.1
BA0: U41.59(A0/ALE) ; also sheet 1,2,5,6,7
BD0: U41.9(PD0) U41.18(BD0) U43.20(B1) ; also sheet 2,5,6,7,10
BD1: U41.8(PD1) U41.17(BD1) U43.19(B2) ; also sheet 2,5,6,7,10
BD2: U41.7(PD2) U41.16(BD2) U43.18(B3) ; also sheet 2,5,6,7,10
BD3: U41.6(PD3) U41.15(BD3) U43.17(B4) ; also sheet 2,5,6,7,10
BD4: U41.5(PD4) U41.14(BD4) U43.16(B5) ; also sheet 2,5,6,7,10
BD5: U41.4(PD5) U41.13(BD5) U43.15(B6) ; also sheet 2,5,6,7
BD6: U41.3(PD6) U41.12(BD6) U43.14(B7) ; also sheet 2,5,6,7
BD7: U41.2(PD7) U41.11(BD7) U43.13(B8) ; also sheet 2,5,6,7
D0: U43.4(A1) ; also sheet 1,8,10
D1: U43.5(A2) ; also sheet 1,8,10
D2: U43.6(A3) ; also sheet 1,8,10
D3: U43.7(A4) ; also sheet 1,8,10
D4: U43.8(A5) ; also sheet 1,8,10
D5: U43.9(A6) ; also sheet 1,8,10
D6: U43.10(A7) ; also sheet 1,8,10
D7: U43.11(A8) ; also sheet 1,8,10
DRQS0: U41.23(BREQ) ; also sheet 2
GND: CONN1.1 CONN1.3 CONN1.5 CONN1.7 CONN1.9 CONN1.11 CONN1.13 CONN1.15 CONN1.17 CONN1.19 CONN1.20 CONN1.21 CONN1.22 CONN1.23 CONN1.24 CONN1.25 CONN1.27 CONN1.28 CONN1.29 CONN1.30 CONN1.31 CONN1.33 CONN1.34 CONN1.35 CONN1.37 CONN1.39 CONN1.41 CONN1.43 CONN1.45 CONN1.47 CONN1.49 RES12.7 RES14.7 U34.7(GND) U41.25(MODE) U41.26(GND) U41.31(GND) U41.37(GND) U41.43(GND) U41.48(GND) U43.1(CAB) U43.2(SAB) U43.12(GND) ; also sheet 1,2,3,5,6,7,8,9,10
PA0: U41.49(PA0) ; also sheet 9
PA1: U41.50(PA1) ; also sheet 9
PA2: U41.51(PA2) ; also sheet 9
PA3: U41.52(PA3) ; also sheet 9
PA4: U41.53(PA4) ; also sheet 9
PA5: U41.54(PA5) ; also sheet 9
PA6: U41.55(PA6) ; also sheet 9
PA7: U41.56(PA7) ; also sheet 9
SCSI0: U41.22(CS) ; also sheet 2
SCSICLK: U34.8(FO) U41.20(!CLK)
STERM0: CONN1.26 D1.C
Unconnected: RES12.1 RES12.8 RES12.9 RES12.10 RES14.8 RES14.9 U34.1(OE) U41.10(BDP) U41.60(PB0) U41.61(PB1) U41.62(PB2) U41.63(PB3) U41.64(PB4) U41.65(PB5) U41.66(PB6) U41.67(PB7) U41.68(PBP)

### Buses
D[0..31]
BD[0..7]

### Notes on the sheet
- (c) 1988,89 George Scolaro
  941 Chehalis Dr.
  Sunnyvale  CA, 94087
- 532 Baby AT
- Buffers & Drive SCSI
- retrotronics.org | n/a | 1D+

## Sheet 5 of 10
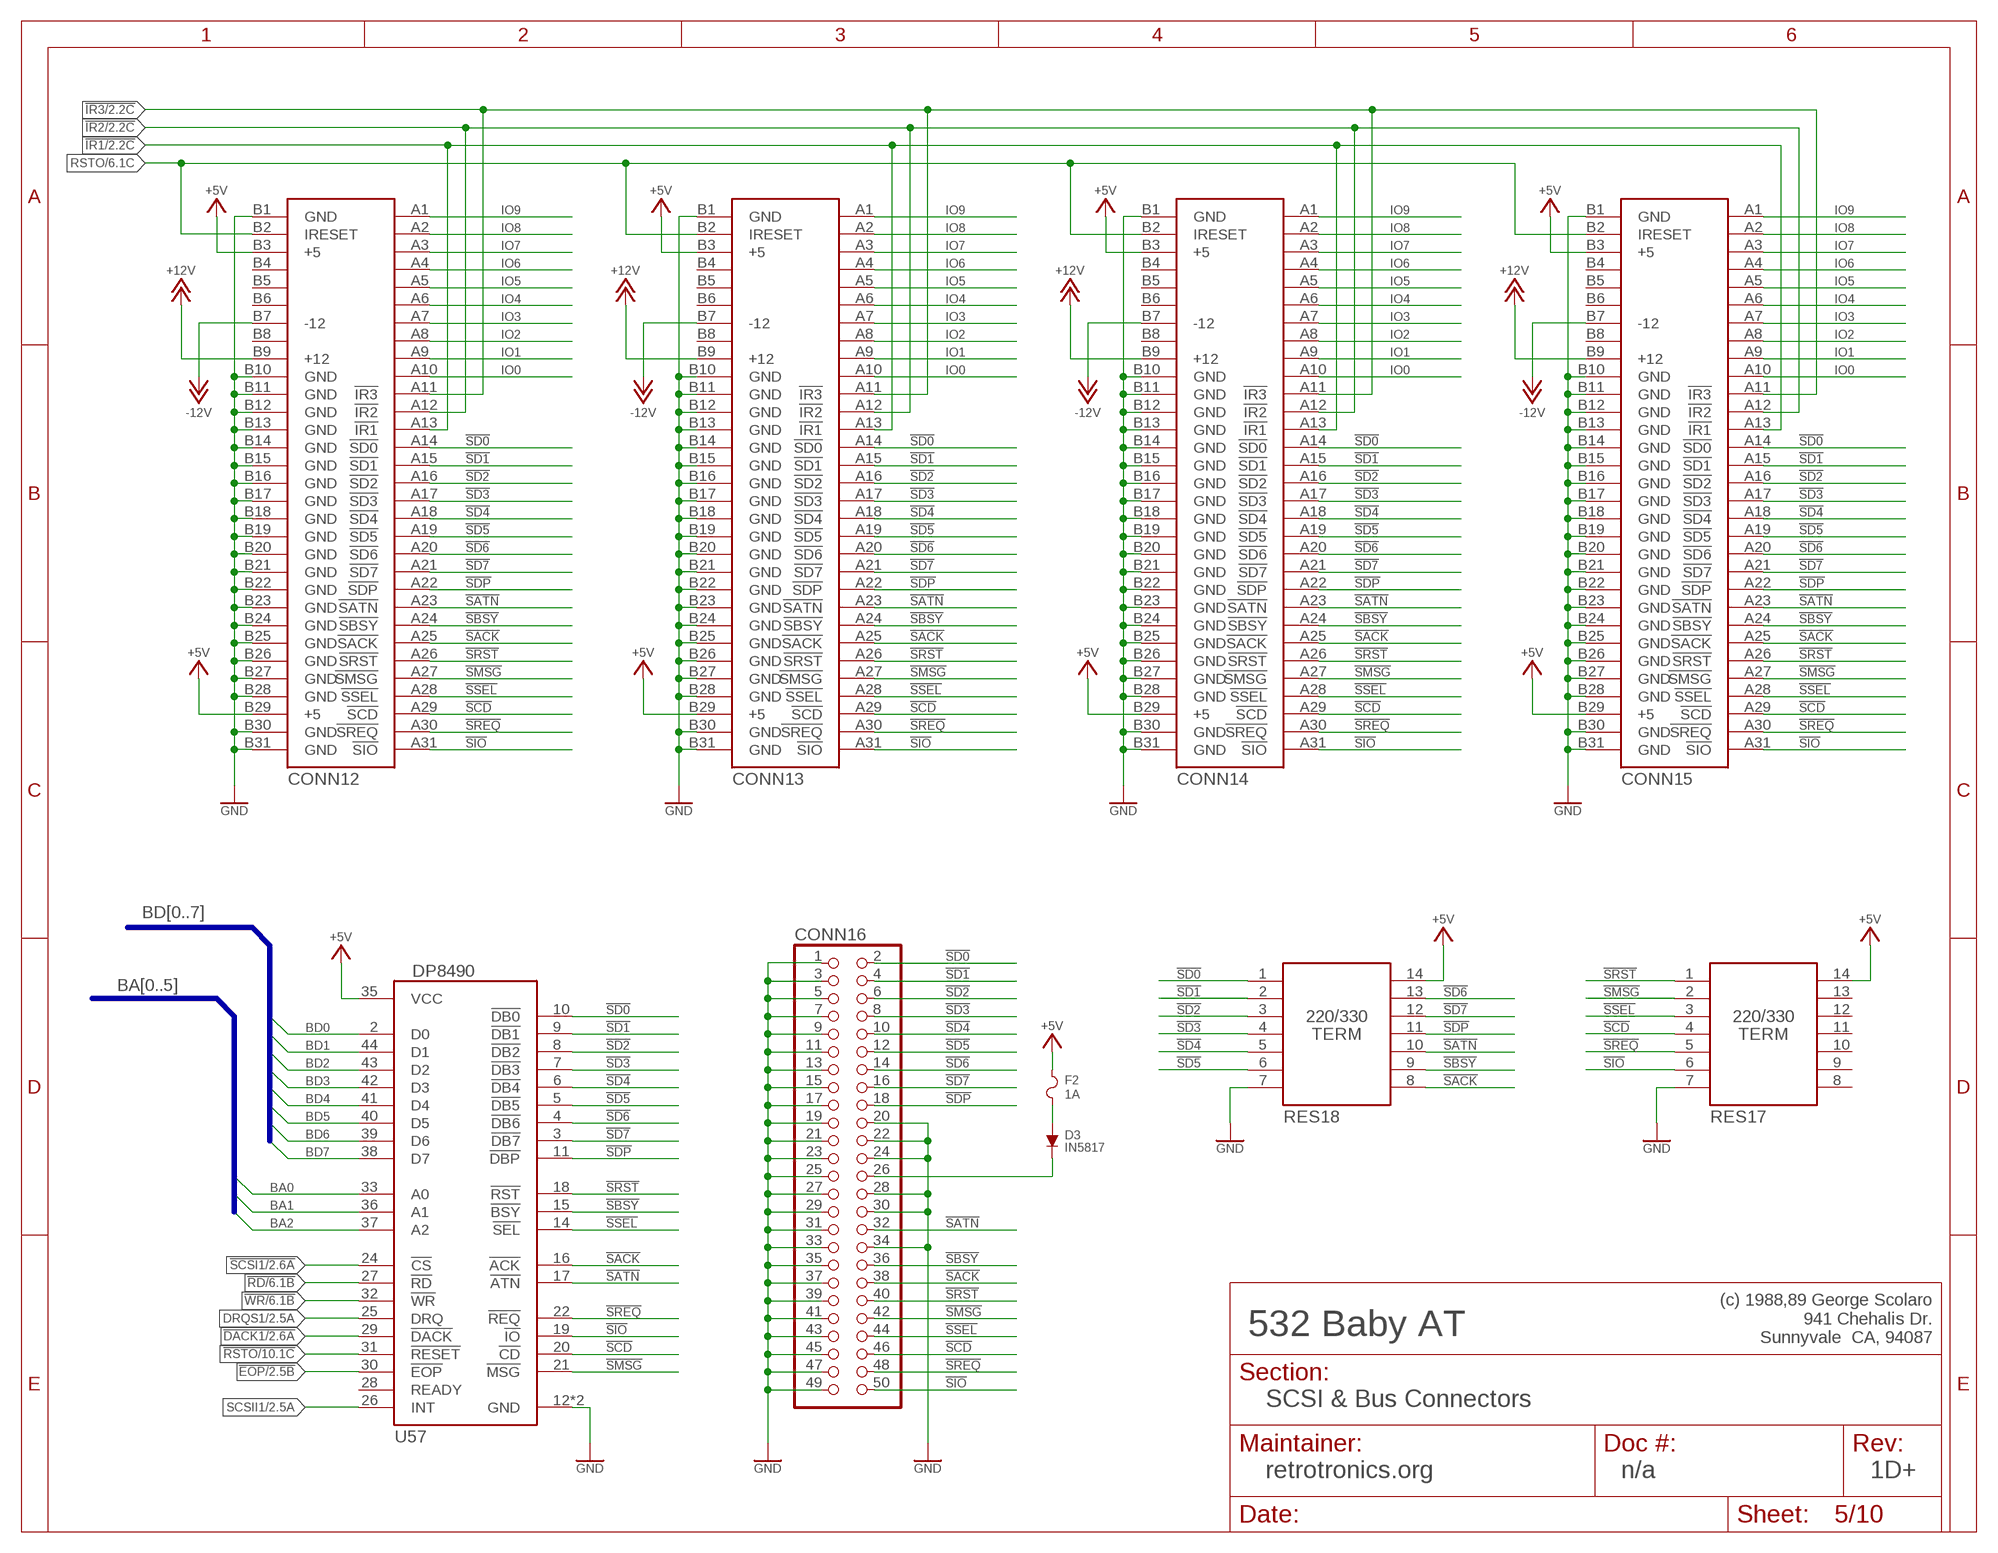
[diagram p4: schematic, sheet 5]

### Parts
CONN12  ISA_SLOT8  [ISA_SLOT8]
CONN13  ISA_SLOT8  [ISA_SLOT8]
CONN14  ISA_SLOT8  [ISA_SLOT8]
CONN15  ISA_SLOT8  [ISA_SLOT8]
CONN16  HDR_2X25  [HDR_2X25]
D3  IN5817  D  [DO35]
F2  1A  FUSE  [FUSE]
RES17  220/330  SCSITERM  [DIL14]
RES18  220/330  SCSITERM  [DIL14]
U57  DP8490  [PLCC44]

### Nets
!DACK1: U57.29(!DACK) ; also sheet 2
!EOP: U57.30(!EOP) ; also sheet 2
!IR1: CONN12.A13(!IR1) CONN13.A13(!IR1) CONN14.A13(!IR1) CONN15.A13(!IR1) ; also sheet 2
!IR2: CONN12.A12(!IR2) CONN13.A12(!IR2) CONN14.A12(!IR2) CONN15.A12(!IR2) ; also sheet 2
!IR3: CONN12.A11(!IR3) CONN13.A11(!IR3) CONN14.A11(!IR3) CONN15.A11(!IR3) ; also sheet 2
!RD: U57.27(!RD) ; also sheet 2,4,6,7,10
!RSTO: U57.31(!RESET) ; also sheet 1,2,4,10
!SACK: CONN12.A25(!SACK) CONN13.A25(!SACK) CONN14.A25(!SACK) CONN15.A25(!SACK) CONN16.38 RES18.8 U57.16(!ACK)
!SATN: CONN12.A23(!SATN) CONN13.A23(!SATN) CONN14.A23(!SATN) CONN15.A23(!SATN) CONN16.32 RES18.10 U57.17(!ATN)
!SBSY: CONN12.A24(!SBSY) CONN13.A24(!SBSY) CONN14.A24(!SBSY) CONN15.A24(!SBSY) CONN16.36 RES18.9 U57.15(!BSY)
!SCD: CONN12.A29(!SCD) CONN13.A29(!SCD) CONN14.A29(!SCD) CONN15.A29(!SCD) CONN16.46 RES17.4 U57.20(!CD)
!SCSI1: U57.24(!CS) ; also sheet 2
!SD0: CONN12.A14(!SD0) CONN13.A14(!SD0) CONN14.A14(!SD0) CONN15.A14(!SD0) CONN16.2 RES18.1 U57.10(!DB0)
!SD1: CONN12.A15(!SD1) CONN13.A15(!SD1) CONN14.A15(!SD1) CONN15.A15(!SD1) CONN16.4 RES18.2 U57.9(!DB1)
!SD2: CONN12.A16(!SD2) CONN13.A16(!SD2) CONN14.A16(!SD2) CONN15.A16(!SD2) CONN16.6 RES18.3 U57.8(!DB2)
!SD3: CONN12.A17(!SD3) CONN13.A17(!SD3) CONN14.A17(!SD3) CONN15.A17(!SD3) CONN16.8 RES18.4 U57.7(!DB3)
!SD4: CONN12.A18(!SD4) CONN13.A18(!SD4) CONN14.A18(!SD4) CONN15.A18(!SD4) CONN16.10 RES18.5 U57.6(!DB4)
!SD5: CONN12.A19(!SD5) CONN13.A19(!SD5) CONN14.A19(!SD5) CONN15.A19(!SD5) CONN16.12 RES18.6 U57.5(!DB5)
!SD6: CONN12.A20(!SD6) CONN13.A20(!SD6) CONN14.A20(!SD6) CONN15.A20(!SD6) CONN16.14 RES18.13 U57.4(!DB6)
!SD7: CONN12.A21(!SD7) CONN13.A21(!SD7) CONN14.A21(!SD7) CONN15.A21(!SD7) CONN16.16 RES18.12 U57.3(!DB7)
!SDP: CONN12.A22(!SDP) CONN13.A22(!SDP) CONN14.A22(!SDP) CONN15.A22(!SDP) CONN16.18 RES18.11 U57.11(!DBP)
!SIO: CONN12.A31(!SIO) CONN13.A31(!SIO) CONN14.A31(!SIO) CONN15.A31(!SIO) CONN16.50 RES17.6 U57.19(!IO)
!SMSG: CONN12.A27(!SMSG) CONN13.A27(!SMSG) CONN14.A27(!SMSG) CONN15.A27(!SMSG) CONN16.42 RES17.2 U57.21(!MSG)
!SREQ: CONN12.A30(!SREQ) CONN13.A30(!SREQ) CONN14.A30(!SREQ) CONN15.A30(!SREQ) CONN16.48 RES17.5 U57.22(!REQ)
!SRST: CONN12.A26(!SRST) CONN13.A26(!SRST) CONN14.A26(!SRST) CONN15.A26(!SRST) CONN16.40 RES17.1 U57.18(!RST)
!SSEL: CONN12.A28(!SSEL) CONN13.A28(!SSEL) CONN14.A28(!SSEL) CONN15.A28(!SSEL) CONN16.44 RES17.3 U57.14(!SEL)
!WR: U57.32(!WR) ; also sheet 2,4,6,7
+5V: CONN12.B3(+5) CONN12.B29(+5) CONN13.B3(+5) CONN13.B29(+5) CONN14.B3(+5) CONN14.B29(+5) CONN15.B3(+5) CONN15.B29(+5) F2.2 RES17.14 RES18.14 U57.35(VCC) ; also sheet 1,2,3,4,6,7,8,9,10
+12V: CONN12.B9(+12) CONN13.B9(+12) CONN14.B9(+12) CONN15.B9(+12) ; also sheet 6,7,9
-12V: CONN12.B7(-12) CONN13.B7(-12) CONN14.B7(-12) CONN15.B7(-12) ; also sheet 6,7,9
_STERM: D3.A F2.1
BA0: U57.33(A0) ; also sheet 1,2,4,6,7
BA1: U57.36(A1) ; also sheet 1,2,6,7
BA2: U57.37(A2) ; also sheet 1,2,6,7
BD0: U57.2(D0) ; also sheet 2,4,6,7,10
BD1: U57.44(D1) ; also sheet 2,4,6,7,10
BD2: U57.43(D2) ; also sheet 2,4,6,7,10
BD3: U57.42(D3) ; also sheet 2,4,6,7,10
BD4: U57.41(D4) ; also sheet 2,4,6,7,10
BD5: U57.40(D5) ; also sheet 2,4,6,7
BD6: U57.39(D6) ; also sheet 2,4,6,7
BD7: U57.38(D7) ; also sheet 2,4,6,7
DRQS1: U57.25(DRQ) ; also sheet 2
GND: CONN12.B1(GND) CONN12.B10(GND) CONN12.B11(GND) CONN12.B12(GND) CONN12.B13(GND) CONN12.B14(GND) CONN12.B15(GND) CONN12.B16(GND) CONN12.B17(GND) CONN12.B18(GND) CONN12.B19(GND) CONN12.B20(GND) CONN12.B21(GND) CONN12.B22(GND) CONN12.B23(GND) CONN12.B24(GND) CONN12.B25(GND) CONN12.B26(GND) CONN12.B27(GND) CONN12.B28(GND) CONN12.B30(GND) CONN12.B31(GND) CONN13.B1(GND) CONN13.B10(GND) CONN13.B11(GND) CONN13.B12(GND) CONN13.B13(GND) CONN13.B14(GND) CONN13.B15(GND) CONN13.B16(GND) CONN13.B17(GND) CONN13.B18(GND) CONN13.B19(GND) CONN13.B20(GND) CONN13.B21(GND) CONN13.B22(GND) CONN13.B23(GND) CONN13.B24(GND) CONN13.B25(GND) CONN13.B26(GND) CONN13.B27(GND) CONN13.B28(GND) CONN13.B30(GND) CONN13.B31(GND) CONN14.B1(GND) CONN14.B10(GND) CONN14.B11(GND) CONN14.B12(GND) CONN14.B13(GND) CONN14.B14(GND) CONN14.B15(GND) CONN14.B16(GND) CONN14.B17(GND) CONN14.B18(GND) CONN14.B19(GND) CONN14.B20(GND) CONN14.B21(GND) CONN14.B22(GND) CONN14.B23(GND) CONN14.B24(GND) CONN14.B25(GND) CONN14.B26(GND) CONN14.B27(GND) CONN14.B28(GND) CONN14.B30(GND) CONN14.B31(GND) CONN15.B1(GND) CONN15.B10(GND) CONN15.B11(GND) CONN15.B12(GND) CONN15.B13(GND) CONN15.B14(GND) CONN15.B15(GND) CONN15.B16(GND) CONN15.B17(GND) CONN15.B18(GND) CONN15.B19(GND) CONN15.B20(GND) CONN15.B21(GND) CONN15.B22(GND) CONN15.B23(GND) CONN15.B24(GND) CONN15.B25(GND) CONN15.B26(GND) CONN15.B27(GND) CONN15.B28(GND) CONN15.B30(GND) CONN15.B31(GND) CONN16.1 CONN16.3 CONN16.5 CONN16.7 CONN16.9 CONN16.11 CONN16.13 CONN16.15 CONN16.17 CONN16.19 CONN16.20 CONN16.21 CONN16.22 CONN16.23 CONN16.24 CONN16.25 CONN16.27 CONN16.28 CONN16.29 CONN16.30 CONN16.31 CONN16.33 CONN16.34 CONN16.35 CONN16.37 CONN16.39 CONN16.41 CONN16.43 CONN16.45 CONN16.47 CONN16.49 RES17.7 RES18.7 U57.12(GND) U57.13(GND) ; also sheet 1,2,3,4,6,7,8,9,10
IO0: CONN12.A10 CONN13.A10 CONN14.A10 CONN15.A10
IO1: CONN12.A9 CONN13.A9 CONN14.A9 CONN15.A9
IO2: CONN12.A8 CONN13.A8 CONN14.A8 CONN15.A8
IO3: CONN12.A7 CONN13.A7 CONN14.A7 CONN15.A7
IO4: CONN12.A6 CONN13.A6 CONN14.A6 CONN15.A6
IO5: CONN12.A5 CONN13.A5 CONN14.A5 CONN15.A5
IO6: CONN12.A4 CONN13.A4 CONN14.A4 CONN15.A4
IO7: CONN12.A3 CONN13.A3 CONN14.A3 CONN15.A3
IO8: CONN12.A2 CONN13.A2 CONN14.A2 CONN15.A2
IO9: CONN12.A1 CONN13.A1 CONN14.A1 CONN15.A1
RSTO: CONN12.B2(IRESET) CONN13.B2(IRESET) CONN14.B2(IRESET) CONN15.B2(IRESET) ; also sheet 6,7,9
SCSII1: U57.26(INT) ; also sheet 2
STERM: CONN16.26 D3.C
Unconnected: CONN12.B4 CONN12.B5 CONN12.B6 CONN12.B8 CONN13.B4 CONN13.B5 CONN13.B6 CONN13.B8 CONN14.B4 CONN14.B5 CONN14.B6 CONN14.B8 CONN15.B4 CONN15.B5 CONN15.B6 CONN15.B8 RES17.8 RES17.9 RES17.10 RES17.11 RES17.12 RES17.13 U57.28(READY)

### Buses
BD[0..7]
BA[0..5]

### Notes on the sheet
- (c) 1988,89 George Scolaro
  941 Chehalis Dr.
  Sunnyvale  CA, 94087
- 532 Baby AT
- SCSI & Bus Connectors
- retrotronics.org | n/a | 1D+

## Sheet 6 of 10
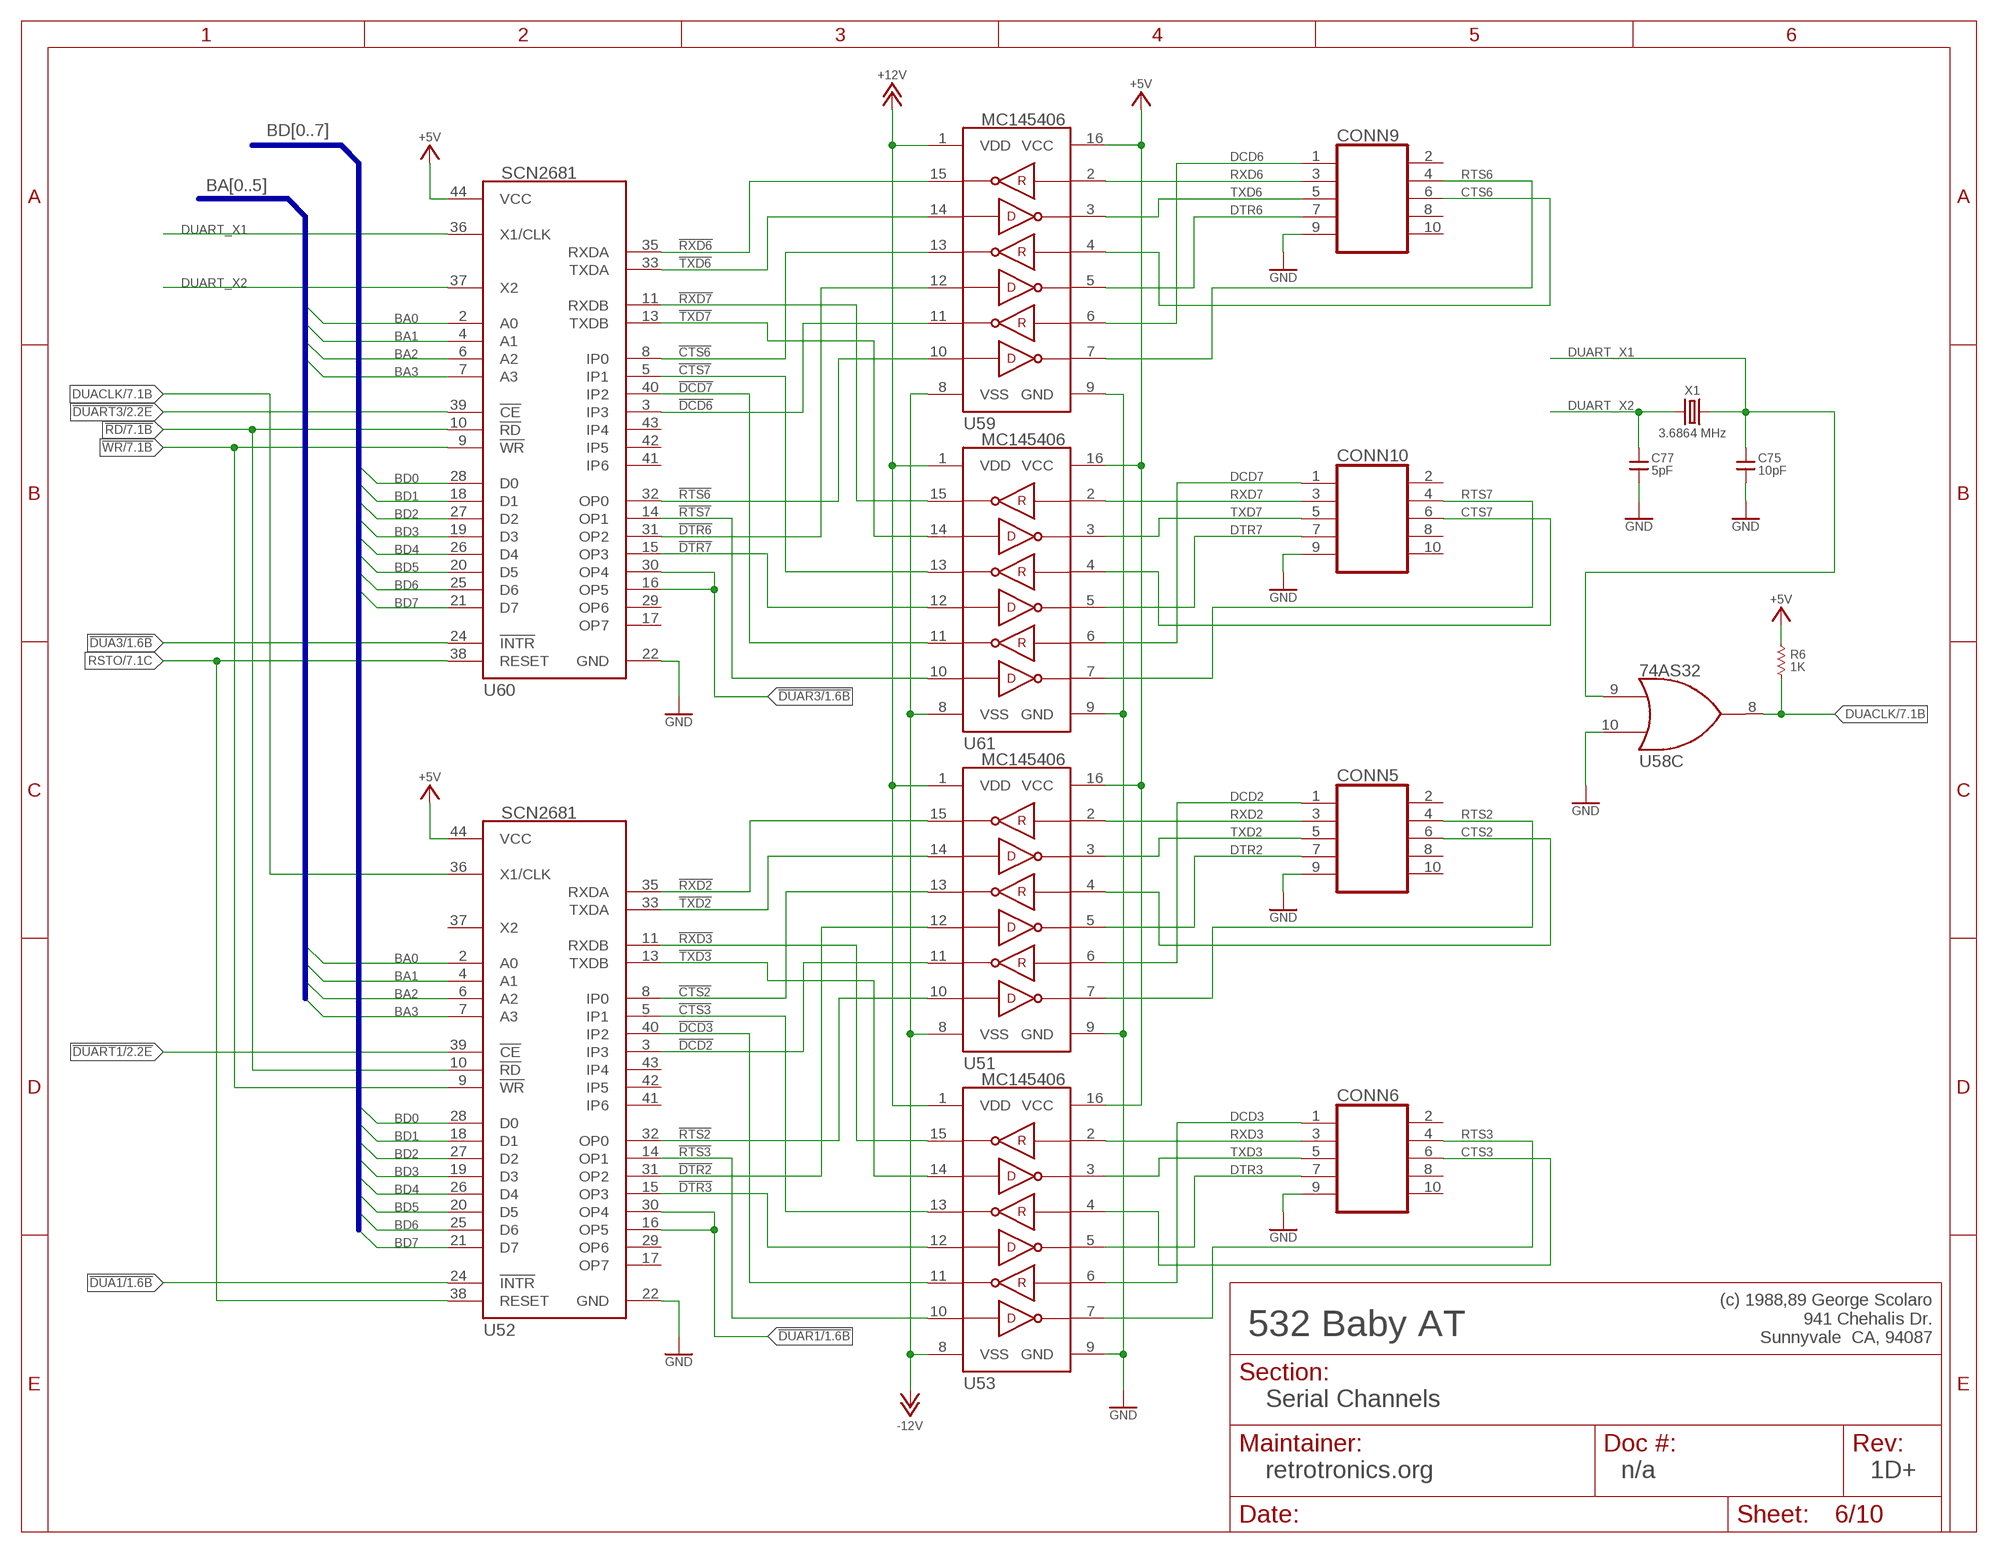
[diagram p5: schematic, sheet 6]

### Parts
C75  10pF  C_US_300M  [C_TH_300MIL]
C77  5pF  C_US_300M  [C_TH_300MIL]
CONN5  HDR_2X5"  [HDR_2X5]
CONN6  HDR_2X5"  [HDR_2X5]
CONN9  HDR_2X5"  [HDR_2X5]
CONN10  HDR_2X5"  [HDR_2X5]
R6  1K  R_US  [R_204/7]
U51  MC145406  [DIL16]
U52  SCN2681  SIGNETICS_SCN2681Q  [PLCC44]
U53  MC145406  [DIL16]
U59  MC145406  [DIL16]
U60  SCN2681  SIGNETICS_SCN2681Q  [PLCC44]
U61  MC145406  [DIL16]
X1  3.6864 MHz  XTAL  [XTAL]

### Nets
!CTS2: U51.13 U52.8(IP0)
!CTS3: U52.5(IP1) U53.13
!CTS6: U59.13 U60.8(IP0)
!CTS7: U60.5(IP1) U61.13
!DCD2: U51.11 U52.3(IP3)
!DCD3: U52.40(IP2) U53.11
!DCD6: U59.11 U60.3(IP3)
!DCD7: U60.40(IP2) U61.11
!DTR2: U51.12 U52.31(OP2)
!DTR3: U52.15(OP3) U53.12
!DTR6: U59.12 U60.31(OP2)
!DTR7: U60.15(OP3) U61.12
!DUA1: U52.24(!INTR) ; also sheet 1,2
!DUA3: U60.24(!INTR) ; also sheet 1,2
!DUAR1: U52.16(OP5) U52.30(OP4) ; also sheet 1,2
!DUAR3: U60.16(OP5) U60.30(OP4) ; also sheet 1,2
!DUART1: U52.39(!CE) ; also sheet 2
!DUART3: U60.39(!CE) ; also sheet 2
!RD: U52.10(!RD) U60.10(!RD) ; also sheet 2,4,5,7,10
!RTS2: U51.10 U52.32(OP0)
!RTS3: U52.14(OP1) U53.10
!RTS6: U59.10 U60.32(OP0)
!RTS7: U60.14(OP1) U61.10
!RXD2: U51.15 U52.35(RXDA)
!RXD3: U52.11(RXDB) U53.15
!RXD6: U59.15 U60.35(RXDA)
!RXD7: U60.11(RXDB) U61.15
!TXD2: U51.14 U52.33(TXDA)
!TXD3: U52.13(TXDB) U53.14
!TXD6: U59.14 U60.33(TXDA)
!TXD7: U60.13(TXDB) U61.14
!WR: U52.9(!WR) U60.9(!WR) ; also sheet 2,4,5,7
+5V: R6.2 U51.16(VCC) U52.44(VCC) U53.16(VCC) U59.16(VCC) U60.44(VCC) U61.16(VCC) ; also sheet 1,2,3,4,5,7,8,9,10
+12V: U51.1(VDD) U53.1(VDD) U59.1(VDD) U61.1(VDD) ; also sheet 5,7,9
-12V: U51.8(VSS) U53.8(VSS) U59.8(VSS) U61.8(VSS) ; also sheet 5,7,9
BA0: U52.2(A0) U60.2(A0) ; also sheet 1,2,4,5,7
BA1: U52.4(A1) U60.4(A1) ; also sheet 1,2,5,7
BA2: U52.6(A2) U60.6(A2) ; also sheet 1,2,5,7
BA3: U52.7(A3) U60.7(A3) ; also sheet 1,2,7
BD0: U52.28(D0) U60.28(D0) ; also sheet 2,4,5,7,10
BD1: U52.18(D1) U60.18(D1) ; also sheet 2,4,5,7,10
BD2: U52.27(D2) U60.27(D2) ; also sheet 2,4,5,7,10
BD3: U52.19(D3) U60.19(D3) ; also sheet 2,4,5,7,10
BD4: U52.26(D4) U60.26(D4) ; also sheet 2,4,5,7,10
BD5: U52.20(D5) U60.20(D5) ; also sheet 2,4,5,7
BD6: U52.25(D6) U60.25(D6) ; also sheet 2,4,5,7
BD7: U52.21(D7) U60.21(D7) ; also sheet 2,4,5,7
CTS2: CONN5.6 U51.4
CTS3: CONN6.6 U53.4
CTS6: CONN9.6 U59.4
CTS7: CONN10.6 U61.4
DCD2: CONN5.1 U51.6
DCD3: CONN6.1 U53.6
DCD6: CONN9.1 U59.6
DCD7: CONN10.1 U61.6
DTR2: CONN5.7 U51.5
DTR3: CONN6.7 U53.5
DTR6: CONN9.7 U59.5
DTR7: CONN10.7 U61.5
DUACLK: R6.1 U52.36(X1/CLK) U58.8(C:Y) ; also sheet 2,7
DUART_X1: C75.1 U58.9(C:A) U60.36(X1/CLK) X1.1
DUART_X2: C77.1 U60.37(X2) X1.2
GND: C75.2 C77.2 CONN5.9 CONN6.9 CONN9.9 CONN10.9 U51.9(GND) U52.22(GND) U53.9(GND) U58.10(C:B) U59.9(GND) U60.22(GND) U61.9(GND) ; also sheet 1,2,3,4,5,7,8,9,10
RSTO: U52.38(RESET) U60.38(RESET) ; also sheet 5,7,9
RTS2: CONN5.4 U51.7
RTS3: CONN6.4 U53.7
RTS6: CONN9.4 U59.7
RTS7: CONN10.4 U61.7
RXD2: CONN5.3 U51.2
RXD3: CONN6.3 U53.2
RXD6: CONN9.3 U59.2
RXD7: CONN10.3 U61.2
TXD2: CONN5.5 U51.3
TXD3: CONN6.5 U53.3
TXD6: CONN9.5 U59.3
TXD7: CONN10.5 U61.3
Unconnected: CONN5.2 CONN5.8 CONN5.10 CONN6.2 CONN6.8 CONN6.10 CONN9.2 CONN9.8 CONN9.10 CONN10.2 CONN10.8 CONN10.10 U52.17(OP7) U52.29(OP6) U52.37(X2) U52.41(IP6) U52.42(IP5) U52.43(IP4) U60.17(OP7) U60.29(OP6) U60.41(IP6) U60.42(IP5) U60.43(IP4)

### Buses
BD[0..7]
BA[0..5]

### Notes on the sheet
- (c) 1988,89 George Scolaro
  941 Chehalis Dr.
  Sunnyvale  CA, 94087
- 532 Baby AT
- Serial Channels
- retrotronics.org | n/a | 1D+

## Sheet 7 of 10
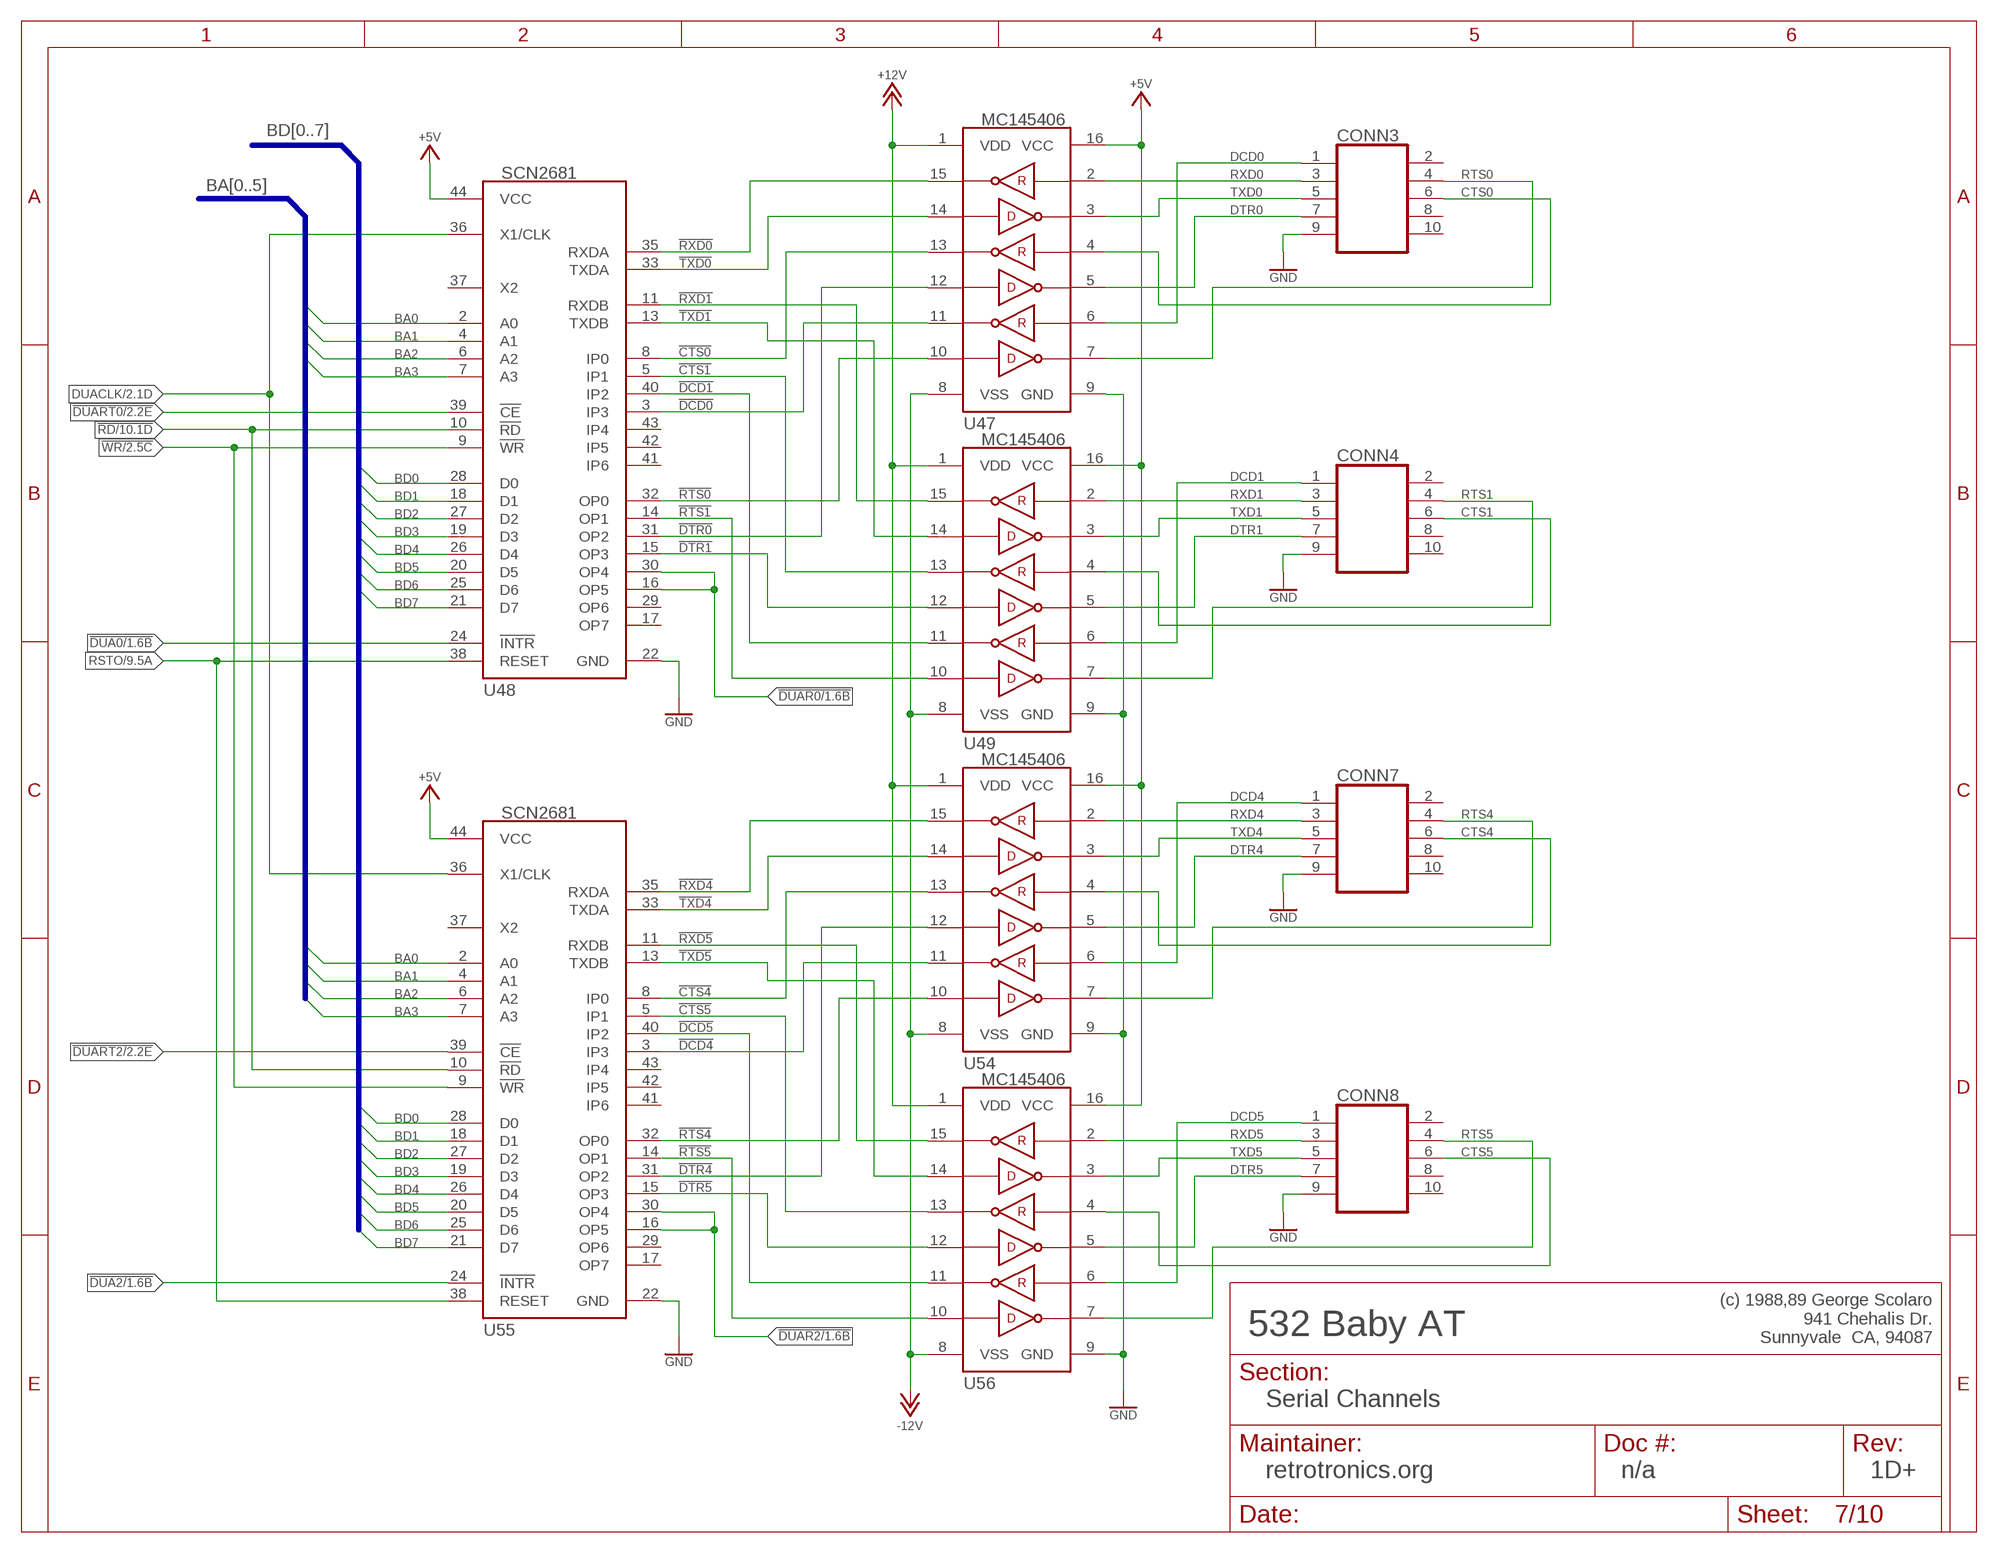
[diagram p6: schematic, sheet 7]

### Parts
CONN3  HDR_2X5"  [HDR_2X5]
CONN4  HDR_2X5"  [HDR_2X5]
CONN7  HDR_2X5"  [HDR_2X5]
CONN8  HDR_2X5"  [HDR_2X5]
U47  MC145406  [DIL16]
U48  SCN2681  SIGNETICS_SCN2681Q  [PLCC44]
U49  MC145406  [DIL16]
U54  MC145406  [DIL16]
U55  SCN2681  SIGNETICS_SCN2681Q  [PLCC44]
U56  MC145406  [DIL16]

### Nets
!CTS0: U47.13 U48.8(IP0)
!CTS1: U48.5(IP1) U49.13
!CTS4: U54.13 U55.8(IP0)
!CTS5: U55.5(IP1) U56.13
!DCD0: U47.11 U48.3(IP3)
!DCD1: U48.40(IP2) U49.11
!DCD4: U54.11 U55.3(IP3)
!DCD5: U55.40(IP2) U56.11
!DTR0: U47.12 U48.31(OP2)
!DTR1: U48.15(OP3) U49.12
!DTR4: U54.12 U55.31(OP2)
!DTR5: U55.15(OP3) U56.12
!DUA0: U48.24(!INTR) ; also sheet 1,2
!DUA2: U55.24(!INTR) ; also sheet 1,2
!DUAR0: U48.16(OP5) U48.30(OP4) ; also sheet 1,2
!DUAR2: U55.16(OP5) U55.30(OP4) ; also sheet 1,2
!DUART0: U48.39(!CE) ; also sheet 2
!DUART2: U55.39(!CE) ; also sheet 2
!RD: U48.10(!RD) U55.10(!RD) ; also sheet 2,4,5,6,10
!RTS0: U47.10 U48.32(OP0)
!RTS1: U48.14(OP1) U49.10
!RTS4: U54.10 U55.32(OP0)
!RTS5: U55.14(OP1) U56.10
!RXD0: U47.15 U48.35(RXDA)
!RXD1: U48.11(RXDB) U49.15
!RXD4: U54.15 U55.35(RXDA)
!RXD5: U55.11(RXDB) U56.15
!TXD0: U47.14 U48.33(TXDA)
!TXD1: U48.13(TXDB) U49.14
!TXD4: U54.14 U55.33(TXDA)
!TXD5: U55.13(TXDB) U56.14
!WR: U48.9(!WR) U55.9(!WR) ; also sheet 2,4,5,6
+5V: U47.16(VCC) U48.44(VCC) U49.16(VCC) U54.16(VCC) U55.44(VCC) U56.16(VCC) ; also sheet 1,2,3,4,5,6,8,9,10
+12V: U47.1(VDD) U49.1(VDD) U54.1(VDD) U56.1(VDD) ; also sheet 5,6,9
-12V: U47.8(VSS) U49.8(VSS) U54.8(VSS) U56.8(VSS) ; also sheet 5,6,9
BA0: U48.2(A0) U55.2(A0) ; also sheet 1,2,4,5,6
BA1: U48.4(A1) U55.4(A1) ; also sheet 1,2,5,6
BA2: U48.6(A2) U55.6(A2) ; also sheet 1,2,5,6
BA3: U48.7(A3) U55.7(A3) ; also sheet 1,2,6
BD0: U48.28(D0) U55.28(D0) ; also sheet 2,4,5,6,10
BD1: U48.18(D1) U55.18(D1) ; also sheet 2,4,5,6,10
BD2: U48.27(D2) U55.27(D2) ; also sheet 2,4,5,6,10
BD3: U48.19(D3) U55.19(D3) ; also sheet 2,4,5,6,10
BD4: U48.26(D4) U55.26(D4) ; also sheet 2,4,5,6,10
BD5: U48.20(D5) U55.20(D5) ; also sheet 2,4,5,6
BD6: U48.25(D6) U55.25(D6) ; also sheet 2,4,5,6
BD7: U48.21(D7) U55.21(D7) ; also sheet 2,4,5,6
CTS0: CONN3.6 U47.4
CTS1: CONN4.6 U49.4
CTS4: CONN7.6 U54.4
CTS5: CONN8.6 U56.4
DCD0: CONN3.1 U47.6
DCD1: CONN4.1 U49.6
DCD4: CONN7.1 U54.6
DCD5: CONN8.1 U56.6
DTR0: CONN3.7 U47.5
DTR1: CONN4.7 U49.5
DTR4: CONN7.7 U54.5
DTR5: CONN8.7 U56.5
DUACLK: U48.36(X1/CLK) U55.36(X1/CLK) ; also sheet 2,6
GND: CONN3.9 CONN4.9 CONN7.9 CONN8.9 U47.9(GND) U48.22(GND) U49.9(GND) U54.9(GND) U55.22(GND) U56.9(GND) ; also sheet 1,2,3,4,5,6,8,9,10
RSTO: U48.38(RESET) U55.38(RESET) ; also sheet 5,6,9
RTS0: CONN3.4 U47.7
RTS1: CONN4.4 U49.7
RTS4: CONN7.4 U54.7
RTS5: CONN8.4 U56.7
RXD0: CONN3.3 U47.2
RXD1: CONN4.3 U49.2
RXD4: CONN7.3 U54.2
RXD5: CONN8.3 U56.2
TXD0: CONN3.5 U47.3
TXD1: CONN4.5 U49.3
TXD4: CONN7.5 U54.3
TXD5: CONN8.5 U56.3
Unconnected: CONN3.2 CONN3.8 CONN3.10 CONN4.2 CONN4.8 CONN4.10 CONN7.2 CONN7.8 CONN7.10 CONN8.2 CONN8.8 CONN8.10 U48.17(OP7) U48.29(OP6) U48.37(X2) U48.41(IP6) U48.42(IP5) U48.43(IP4) U55.17(OP7) U55.29(OP6) U55.37(X2) U55.41(IP6) U55.42(IP5) U55.43(IP4)

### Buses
BD[0..7]
BA[0..5]

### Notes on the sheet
- (c) 1988,89 George Scolaro
  941 Chehalis Dr.
  Sunnyvale  CA, 94087
- 532 Baby AT
- Serial Channels
- retrotronics.org | n/a | 1D+

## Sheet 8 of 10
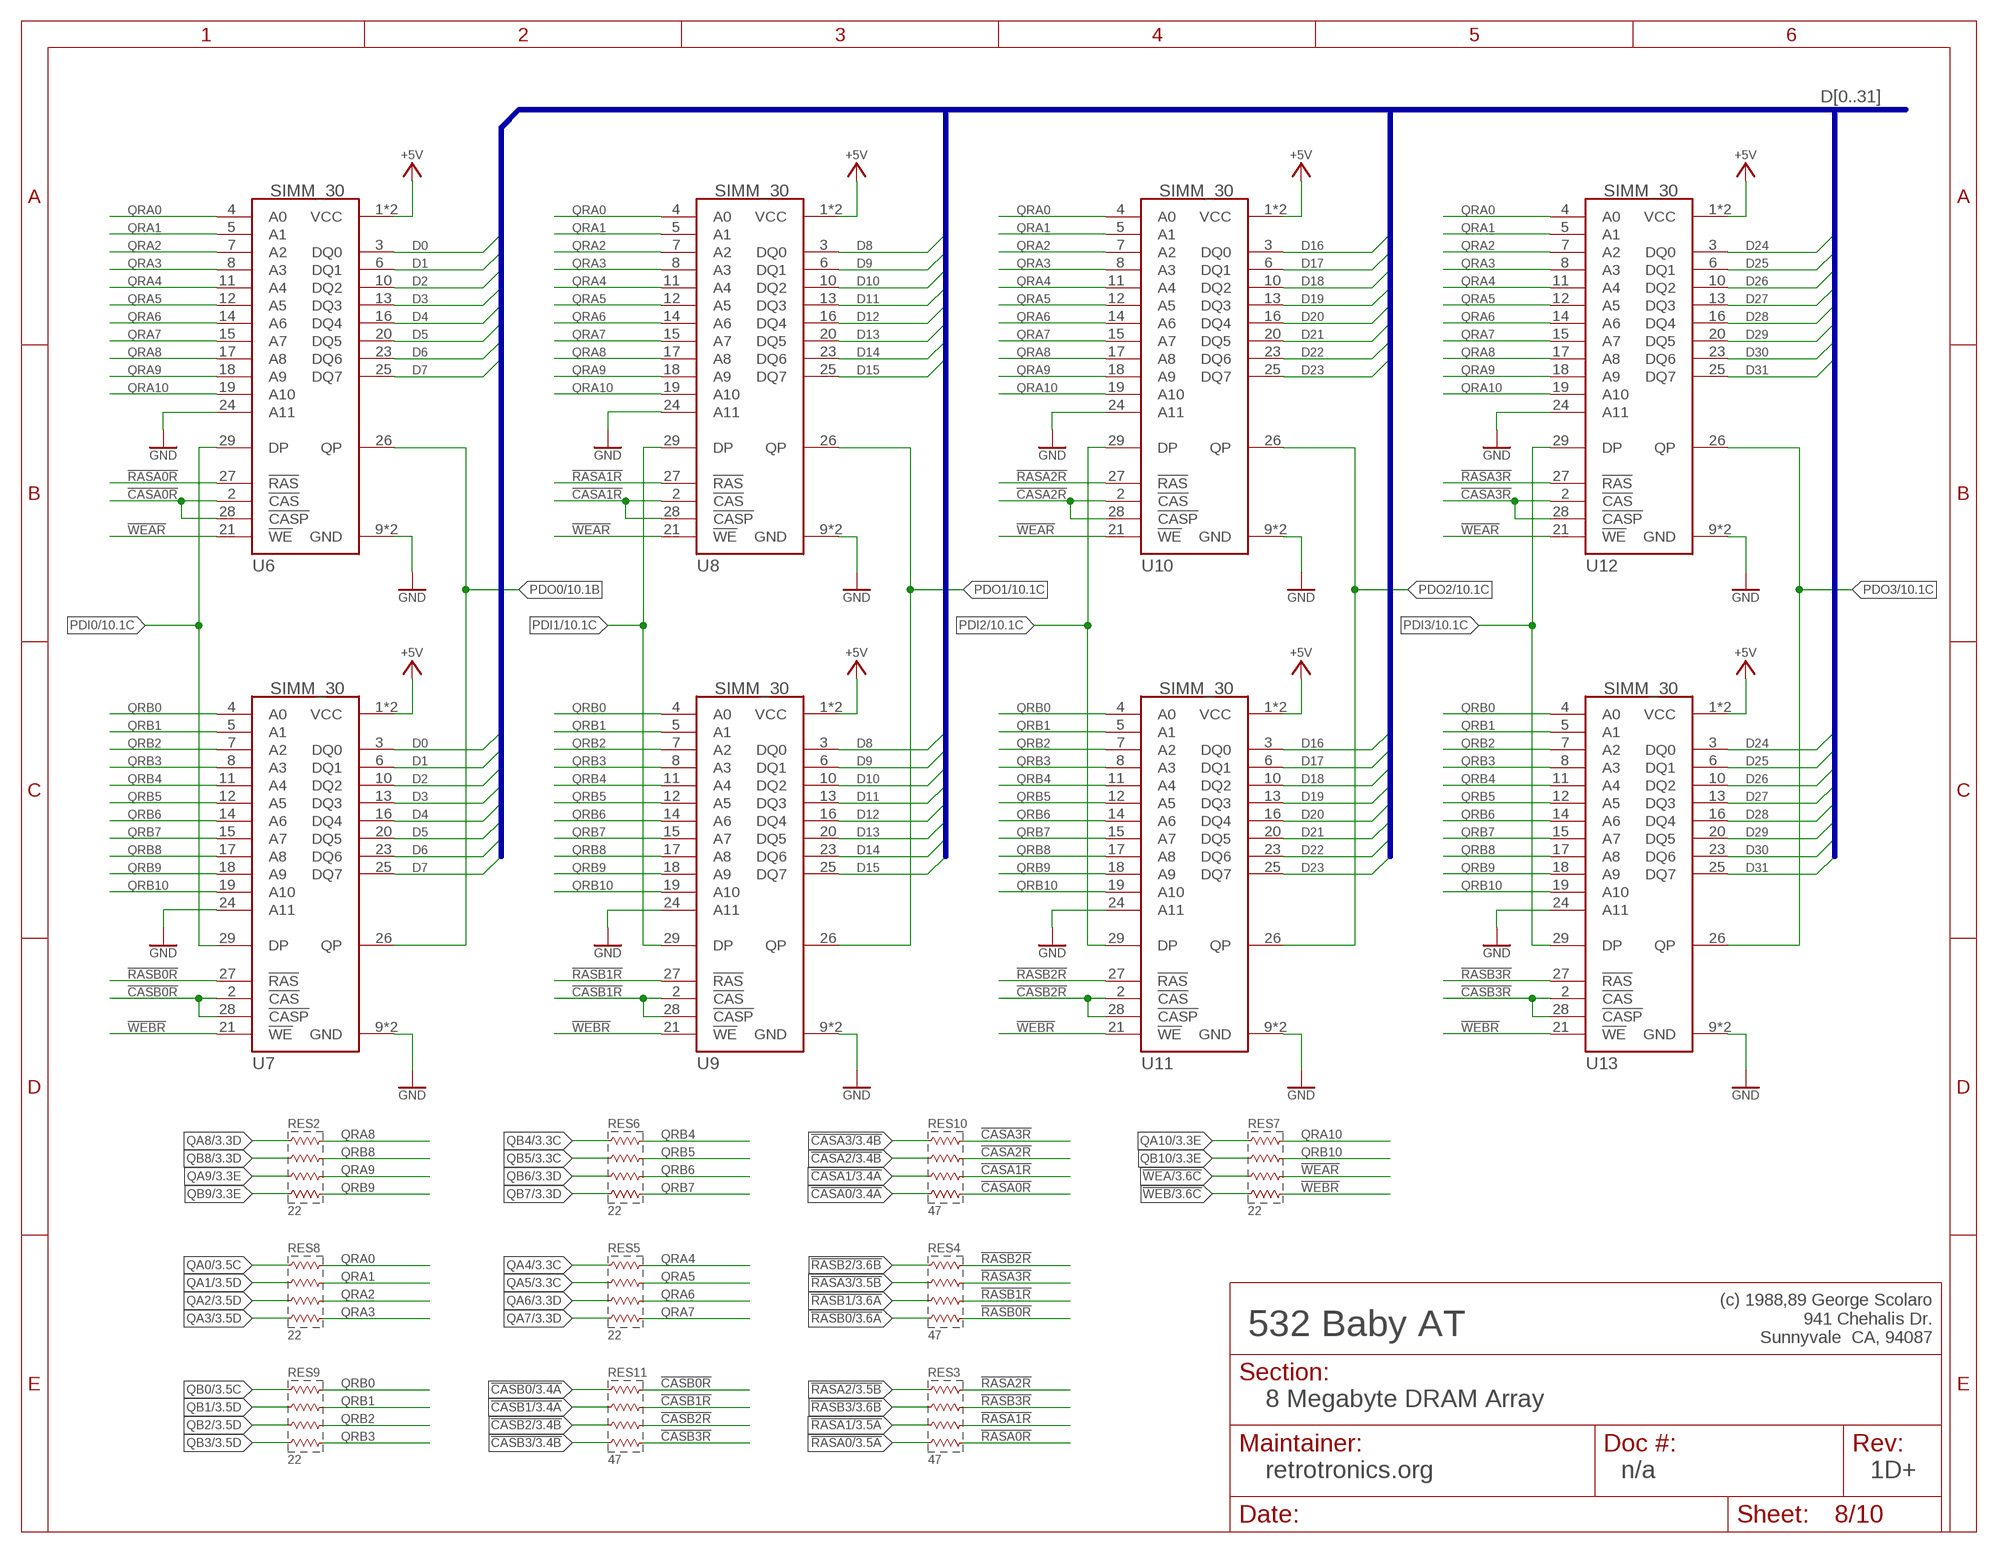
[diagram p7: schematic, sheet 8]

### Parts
RES2  22  RA_SIP_X4  [RN_SIP8]
RES3  47  RA_SIP_X4  [RN_SIP8]
RES4  47  RA_SIP_X4  [RN_SIP8]
RES5  22  RA_SIP_X4  [RN_SIP8]
RES6  22  RA_SIP_X4  [RN_SIP8]
RES7  22  RA_SIP_X4  [RN_SIP8]
RES8  22  RA_SIP_X4  [RN_SIP8]
RES9  22  RA_SIP_X4  [RN_SIP8]
RES10  47  RA_SIP_X4  [RN_SIP8]
RES11  47  RA_SIP_X4  [RN_SIP8]
U6  SIMM_30  [SIMM_30]
U7  SIMM_30  [SIMM_30]
U8  SIMM_30  [SIMM_30]
U9  SIMM_30  [SIMM_30]
U10  SIMM_30  [SIMM_30]
U11  SIMM_30  [SIMM_30]
U12  SIMM_30  [SIMM_30]
U13  SIMM_30  [SIMM_30]

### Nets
!CASA0: RES10.7 ; also sheet 3
!CASA0R: RES10.8 U6.2(!CAS) U6.28(!CASP)
!CASA1: RES10.5 ; also sheet 3
!CASA1R: RES10.6 U8.2(!CAS) U8.28(!CASP)
!CASA2: RES10.3 ; also sheet 3
!CASA2R: RES10.4 U10.2(!CAS) U10.28(!CASP)
!CASA3: RES10.1 ; also sheet 3
!CASA3R: RES10.2 U12.2(!CAS) U12.28(!CASP)
!CASB0: RES11.1 ; also sheet 3
!CASB0R: RES11.2 U7.2(!CAS) U7.28(!CASP)
!CASB1: RES11.3 ; also sheet 3
!CASB1R: RES11.4 U9.2(!CAS) U9.28(!CASP)
!CASB2: RES11.5 ; also sheet 3
!CASB2R: RES11.6 U11.2(!CAS) U11.28(!CASP)
!CASB3: RES11.7 ; also sheet 3
!CASB3R: RES11.8 U13.2(!CAS) U13.28(!CASP)
!RASA0: RES3.7 ; also sheet 3
!RASA0R: RES3.8 U6.27(!RAS)
!RASA1: RES3.5 ; also sheet 3
!RASA1R: RES3.6 U8.27(!RAS)
!RASA2: RES3.1 ; also sheet 3
!RASA2R: RES3.2 U10.27(!RAS)
!RASA3: RES4.3 ; also sheet 3
!RASA3R: RES4.4 U12.27(!RAS)
!RASB0: RES4.7 ; also sheet 3
!RASB0R: RES4.8 U7.27(!RAS)
!RASB1: RES4.5 ; also sheet 3
!RASB1R: RES4.6 U9.27(!RAS)
!RASB2: RES4.1 ; also sheet 3
!RASB2R: RES4.2 U11.27(!RAS)
!RASB3: RES3.3 ; also sheet 3
!RASB3R: RES3.4 U13.27(!RAS)
!WEA: RES7.5 ; also sheet 3
!WEAR: RES7.6 U6.21(!WE) U8.21(!WE) U10.21(!WE) U12.21(!WE)
!WEB: RES7.7 ; also sheet 3
!WEBR: RES7.8 U7.21(!WE) U9.21(!WE) U11.21(!WE) U13.21(!WE)
+5V: U6.1(VCC) U6.30(VCC) U7.1(VCC) U7.30(VCC) U8.1(VCC) U8.30(VCC) U9.1(VCC) U9.30(VCC) U10.1(VCC) U10.30(VCC) U11.1(VCC) U11.30(VCC) U12.1(VCC) U12.30(VCC) U13.1(VCC) U13.30(VCC) ; also sheet 1,2,3,4,5,6,7,9,10
D0: U6.3(DQ0) U7.3(DQ0) ; also sheet 1,4,10
D1: U6.6(DQ1) U7.6(DQ1) ; also sheet 1,4,10
D2: U6.10(DQ2) U7.10(DQ2) ; also sheet 1,4,10
D3: U6.13(DQ3) U7.13(DQ3) ; also sheet 1,4,10
D4: U6.16(DQ4) U7.16(DQ4) ; also sheet 1,4,10
D5: U6.20(DQ5) U7.20(DQ5) ; also sheet 1,4,10
D6: U6.23(DQ6) U7.23(DQ6) ; also sheet 1,4,10
D7: U6.25(DQ7) U7.25(DQ7) ; also sheet 1,4,10
D8: U8.3(DQ0) U9.3(DQ0) ; also sheet 1,10
D9: U8.6(DQ1) U9.6(DQ1) ; also sheet 1,10
D10: U8.10(DQ2) U9.10(DQ2) ; also sheet 1,10
D11: U8.13(DQ3) U9.13(DQ3) ; also sheet 1,10
D12: U8.16(DQ4) U9.16(DQ4) ; also sheet 1,10
D13: U8.20(DQ5) U9.20(DQ5) ; also sheet 1,10
D14: U8.23(DQ6) U9.23(DQ6) ; also sheet 1,10
D15: U8.25(DQ7) U9.25(DQ7) ; also sheet 1,10
D16: U10.3(DQ0) U11.3(DQ0) ; also sheet 1,10
D17: U10.6(DQ1) U11.6(DQ1) ; also sheet 1,10
D18: U10.10(DQ2) U11.10(DQ2) ; also sheet 1,10
D19: U10.13(DQ3) U11.13(DQ3) ; also sheet 1,10
D20: U10.16(DQ4) U11.16(DQ4) ; also sheet 1,10
D21: U10.20(DQ5) U11.20(DQ5) ; also sheet 1,10
D22: U10.23(DQ6) U11.23(DQ6) ; also sheet 1,10
D23: U10.25(DQ7) U11.25(DQ7) ; also sheet 1,10
D24: U12.3(DQ0) U13.3(DQ0) ; also sheet 1,10
D25: U12.6(DQ1) U13.6(DQ1) ; also sheet 1,10
D26: U12.10(DQ2) U13.10(DQ2) ; also sheet 1,10
D27: U12.13(DQ3) U13.13(DQ3) ; also sheet 1,10
D28: U12.16(DQ4) U13.16(DQ4) ; also sheet 1,10
D29: U12.20(DQ5) U13.20(DQ5) ; also sheet 1,10
D30: U12.23(DQ6) U13.23(DQ6) ; also sheet 1,10
D31: U12.25(DQ7) U13.25(DQ7) ; also sheet 1,10
GND: U6.9(GND) U6.22(GND) U6.24(A11) U7.9(GND) U7.22(GND) U7.24(A11) U8.9(GND) U8.22(GND) U8.24(A11) U9.9(GND) U9.22(GND) U9.24(A11) U10.9(GND) U10.22(GND) U10.24(A11) U11.9(GND) U11.22(GND) U11.24(A11) U12.9(GND) U12.22(GND) U12.24(A11) U13.9(GND) U13.22(GND) U13.24(A11) ; also sheet 1,2,3,4,5,6,7,9,10
PDI0: U6.29(DP) U7.29(DP) ; also sheet 10
PDI1: U8.29(DP) U9.29(DP) ; also sheet 10
PDI2: U10.29(DP) U11.29(DP) ; also sheet 10
PDI3: U12.29(DP) U13.29(DP) ; also sheet 10
PDO0: U6.26(QP) U7.26(QP) ; also sheet 10
PDO1: U8.26(QP) U9.26(QP) ; also sheet 10
PDO2: U10.26(QP) U11.26(QP) ; also sheet 10
PDO3: U12.26(QP) U13.26(QP) ; also sheet 10
QA0: RES8.1 ; also sheet 3
QA1: RES8.3 ; also sheet 3
QA2: RES8.5 ; also sheet 3
QA3: RES8.7 ; also sheet 3
QA4: RES5.1 ; also sheet 3
QA5: RES5.3 ; also sheet 3
QA6: RES5.5 ; also sheet 3
QA7: RES5.7 ; also sheet 3
QA8: RES2.1 ; also sheet 3
QA9: RES2.5 ; also sheet 3
QA10: RES7.1 ; also sheet 3
QB0: RES9.1 ; also sheet 3
QB1: RES9.3 ; also sheet 3
QB2: RES9.5 ; also sheet 3
QB3: RES9.7 ; also sheet 3
QB4: RES6.1 ; also sheet 3
QB5: RES6.3 ; also sheet 3
QB6: RES6.5 ; also sheet 3
QB7: RES6.7 ; also sheet 3
QB8: RES2.3 ; also sheet 3
QB9: RES2.7 ; also sheet 3
QB10: RES7.3 ; also sheet 3
QRA0: RES8.2 U6.4(A0) U8.4(A0) U10.4(A0) U12.4(A0)
QRA1: RES8.4 U6.5(A1) U8.5(A1) U10.5(A1) U12.5(A1)
QRA2: RES8.6 U6.7(A2) U8.7(A2) U10.7(A2) U12.7(A2)
QRA3: RES8.8 U6.8(A3) U8.8(A3) U10.8(A3) U12.8(A3)
QRA4: RES5.2 U6.11(A4) U8.11(A4) U10.11(A4) U12.11(A4)
QRA5: RES5.4 U6.12(A5) U8.12(A5) U10.12(A5) U12.12(A5)
QRA6: RES5.6 U6.14(A6) U8.14(A6) U10.14(A6) U12.14(A6)
QRA7: RES5.8 U6.15(A7) U8.15(A7) U10.15(A7) U12.15(A7)
QRA8: RES2.2 U6.17(A8) U8.17(A8) U10.17(A8) U12.17(A8)
QRA9: RES2.6 U6.18(A9) U8.18(A9) U10.18(A9) U12.18(A9)
QRA10: RES7.2 U6.19(A10) U8.19(A10) U10.19(A10) U12.19(A10)
QRB0: RES9.2 U7.4(A0) U9.4(A0) U11.4(A0) U13.4(A0)
QRB1: RES9.4 U7.5(A1) U9.5(A1) U11.5(A1) U13.5(A1)
QRB2: RES9.6 U7.7(A2) U9.7(A2) U11.7(A2) U13.7(A2)
QRB3: RES9.8 U7.8(A3) U9.8(A3) U11.8(A3) U13.8(A3)
QRB4: RES6.2 U7.11(A4) U9.11(A4) U11.11(A4) U13.11(A4)
QRB5: RES6.4 U7.12(A5) U9.12(A5) U11.12(A5) U13.12(A5)
QRB6: RES6.6 U7.14(A6) U9.14(A6) U11.14(A6) U13.14(A6)
QRB7: RES6.8 U7.15(A7) U9.15(A7) U11.15(A7) U13.15(A7)
QRB8: RES2.4 U7.17(A8) U9.17(A8) U11.17(A8) U13.17(A8)
QRB9: RES2.8 U7.18(A9) U9.18(A9) U11.18(A9) U13.18(A9)
QRB10: RES7.4 U7.19(A10) U9.19(A10) U11.19(A10) U13.19(A10)

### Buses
D[0..31]

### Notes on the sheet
- (c) 1988,89 George Scolaro
  941 Chehalis Dr.
  Sunnyvale  CA, 94087
- 532 Baby AT
- 8 Megabyte DRAM Array
- retrotronics.org | n/a | 1D+

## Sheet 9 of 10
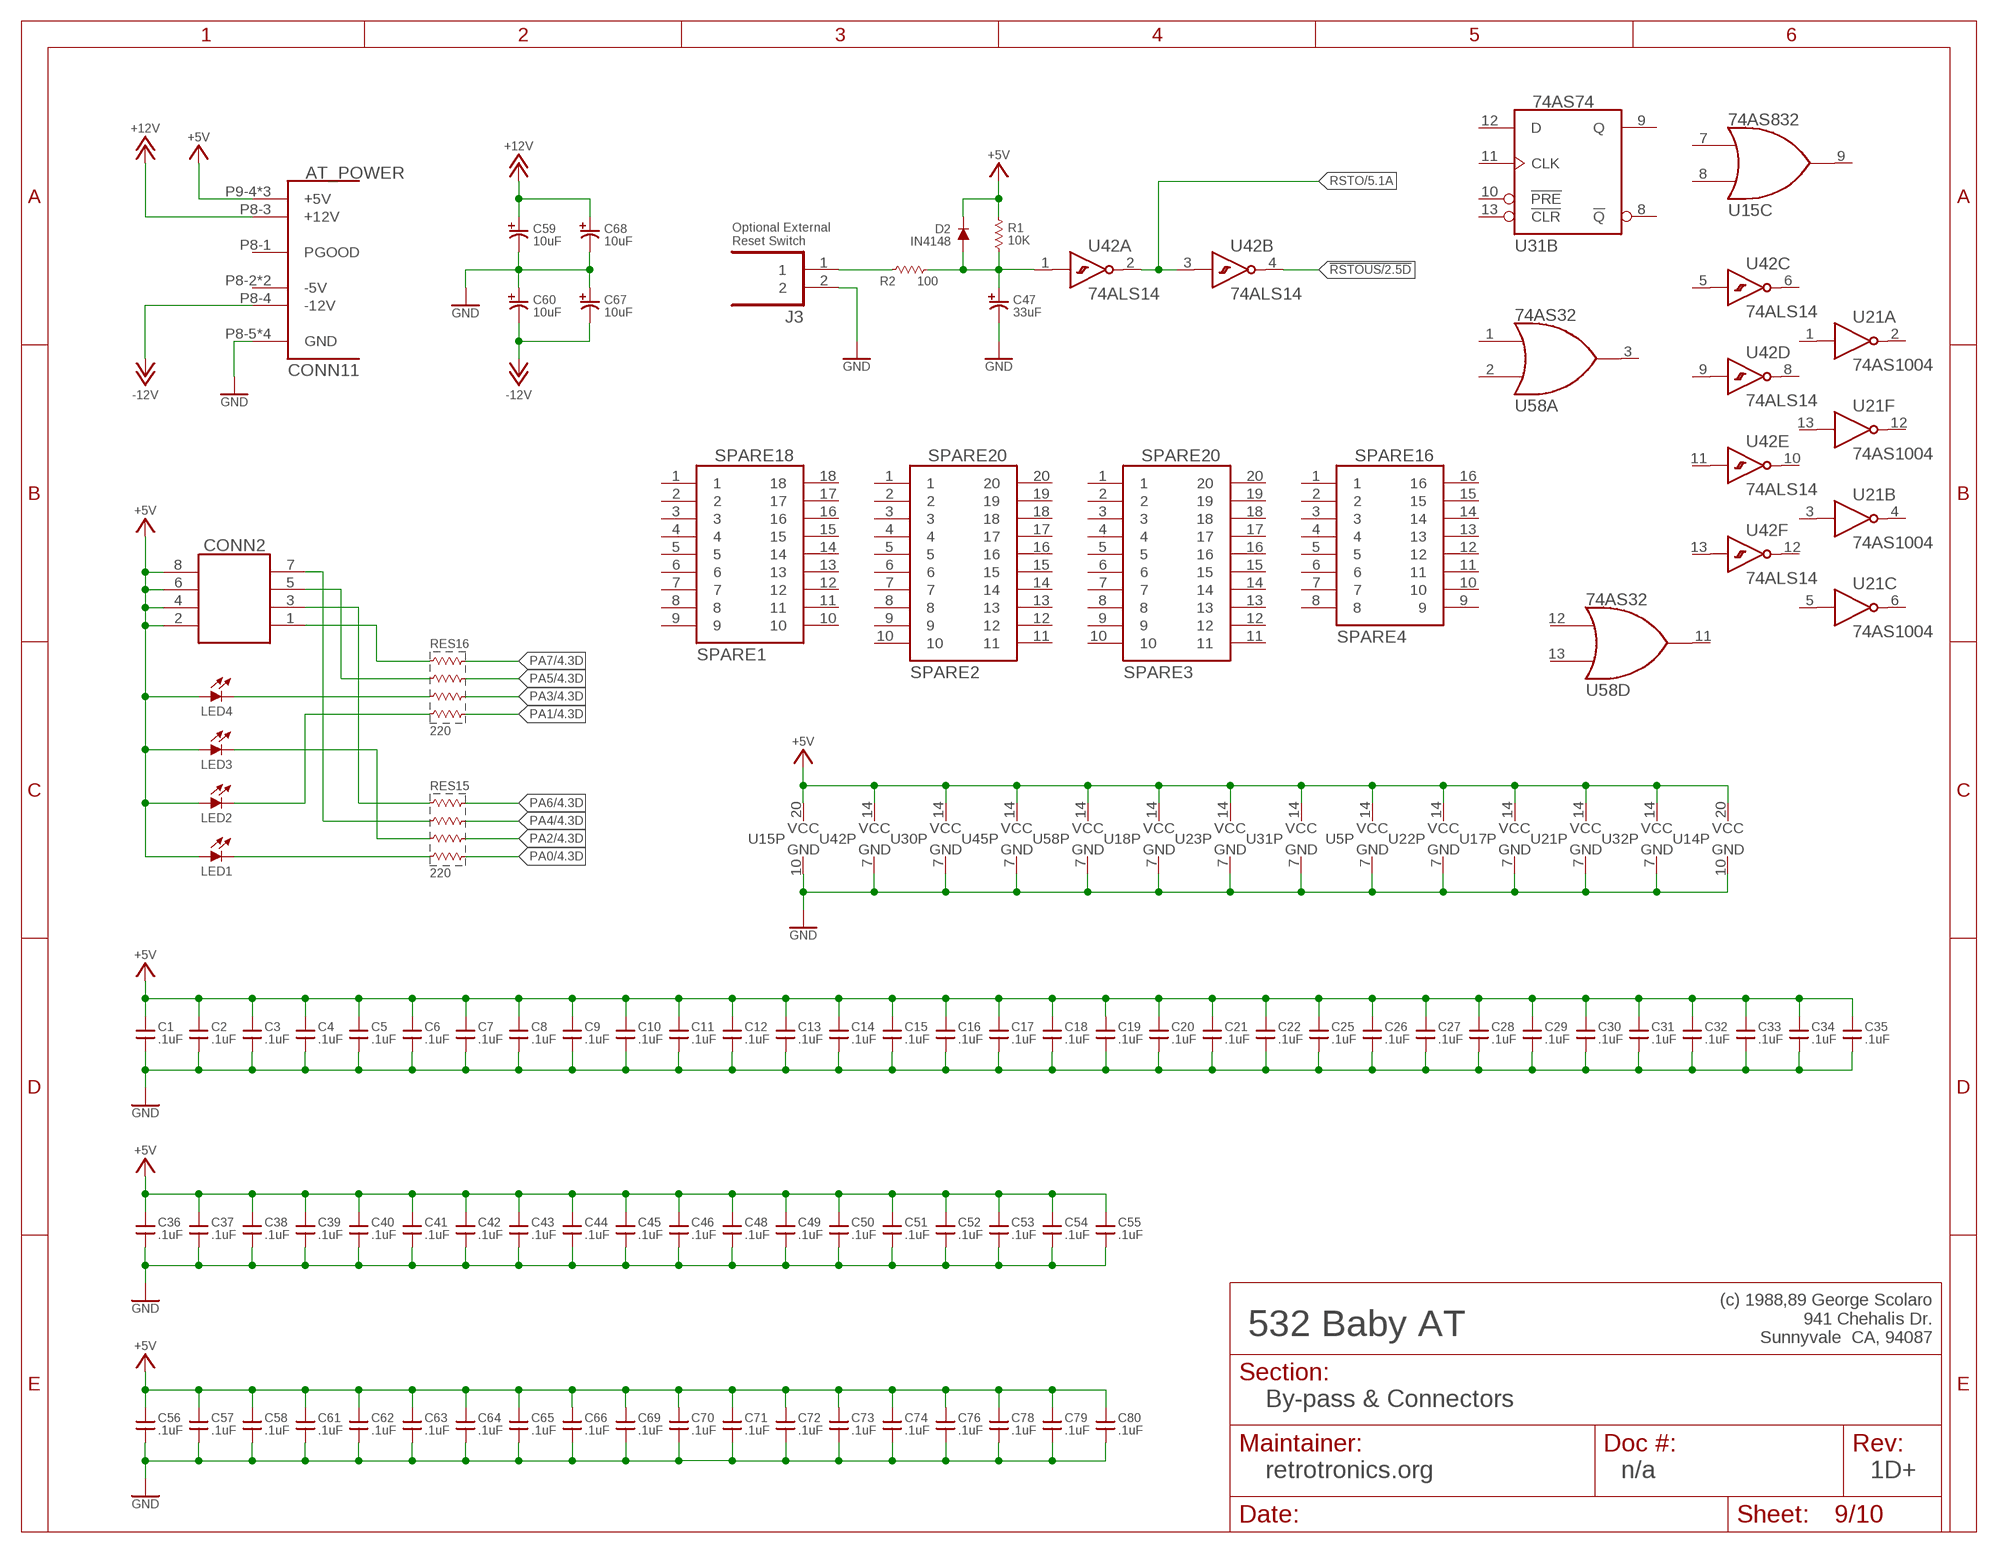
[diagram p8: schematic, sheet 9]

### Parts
C1  .1uF  C_US_300M  [C_TH_300MIL]
C2  .1uF  C_US_300M  [C_TH_300MIL]
C3  .1uF  C_US_300M  [C_TH_300MIL]
C4  .1uF  C_US_300M  [C_TH_300MIL]
C5  .1uF  C_US_300M  [C_TH_300MIL]
C6  .1uF  C_US_300M  [C_TH_300MIL]
C7  .1uF  C_US_300M  [C_TH_300MIL]
C8  .1uF  C_US_300M  [C_TH_300MIL]
C9  .1uF  C_US_300M  [C_TH_300MIL]
C10  .1uF  C_US_300M  [C_TH_300MIL]
C11  .1uF  C_US_300M  [C_TH_300MIL]
C12  .1uF  C_US_300M  [C_TH_300MIL]
C13  .1uF  C_US_300M  [C_TH_300MIL]
C14  .1uF  C_US_300M  [C_TH_300MIL]
C15  .1uF  C_US_300M  [C_TH_300MIL]
C16  .1uF  C_US_300M  [C_TH_300MIL]
C17  .1uF  C_US_300M  [C_TH_300MIL]
C18  .1uF  C_US_300M  [C_TH_300MIL]
C19  .1uF  C_US_300M  [C_TH_300MIL]
C20  .1uF  C_US_300M  [C_TH_300MIL]
C21  .1uF  C_US_300M  [C_TH_300MIL]
C22  .1uF  C_US_300M  [C_TH_300MIL]
C25  .1uF  C_US_300M  [C_TH_300MIL]
C26  .1uF  C_US_300M  [C_TH_300MIL]
C27  .1uF  C_US_300M  [C_TH_300MIL]
C28  .1uF  C_US_300M  [C_TH_300MIL]
C29  .1uF  C_US_300M  [C_TH_300MIL]
C30  .1uF  C_US_300M  [C_TH_300MIL]
C31  .1uF  C_US_300M  [C_TH_300MIL]
C32  .1uF  C_US_300M  [C_TH_300MIL]
C33  .1uF  C_US_300M  [C_TH_300MIL]
C34  .1uF  C_US_300M  [C_TH_300MIL]
C35  .1uF  C_US_300M  [C_TH_300MIL]
C36  .1uF  C_US_300M  [C_TH_300MIL]
C37  .1uF  C_US_300M  [C_TH_300MIL]
C38  .1uF  C_US_300M  [C_TH_300MIL]
C39  .1uF  C_US_300M  [C_TH_300MIL]
C40  .1uF  C_US_300M  [C_TH_300MIL]
C41  .1uF  C_US_300M  [C_TH_300MIL]
C42  .1uF  C_US_300M  [C_TH_300MIL]
C43  .1uF  C_US_300M  [C_TH_300MIL]
C44  .1uF  C_US_300M  [C_TH_300MIL]
C45  .1uF  C_US_300M  [C_TH_300MIL]
C46  .1uF  C_US_300M  [C_TH_300MIL]
C47  33uF  C_POL_US  [C_CYL_5X4MX]
C48  .1uF  C_US_300M  [C_TH_300MIL]
C49  .1uF  C_US_300M  [C_TH_300MIL]
C50  .1uF  C_US_300M  [C_TH_300MIL]
C51  .1uF  C_US_300M  [C_TH_300MIL]
C52  .1uF  C_US_300M  [C_TH_300MIL]
C53  .1uF  C_US_300M  [C_TH_300MIL]
C54  .1uF  C_US_300M  [C_TH_300MIL]
C55  .1uF  C_US_300M  [C_TH_300MIL]
C56  .1uF  C_US_300M  [C_TH_300MIL]
C57  .1uF  C_US_300M  [C_TH_300MIL]
C58  .1uF  C_US_300M  [C_TH_300MIL]
C59  10uF  C_POL_US  [C_CYL_5X4MX]
C60  10uF  C_POL_US  [C_CYL_5X4MX]
C61  .1uF  C_US_300M  [C_TH_300MIL]
C62  .1uF  C_US_300M  [C_TH_300MIL]
C63  .1uF  C_US_300M  [C_TH_300MIL]
C64  .1uF  C_US_300M  [C_TH_300MIL]
C65  .1uF  C_US_300M  [C_TH_300MIL]
C66  .1uF  C_US_300M  [C_TH_300MIL]
C67  10uF  C_POL_US  [C_CYL_5X4MX]
C68  10uF  C_POL_US  [C_CYL_5X4MX]
C69  .1uF  C_US_300M  [C_TH_300MIL]
C70  .1uF  C_US_300M  [C_TH_300MIL]
C71  .1uF  C_US_300M  [C_TH_300MIL]
C72  .1uF  C_US_300M  [C_TH_300MIL]
C73  .1uF  C_US_300M  [C_TH_300MIL]
C74  .1uF  C_US_300M  [C_TH_300MIL]
C76  .1uF  C_US_300M  [C_TH_300MIL]
C78  .1uF  C_US_300M  [C_TH_300MIL]
C79  .1uF  C_US_300M  [C_TH_300MIL]
C80  .1uF  C_US_300M  [C_TH_300MIL]
CONN2  HDR_2X4  [HDR_2X5]
CONN11  AT_POWER  [AT_POWER]
D2  IN4148  D  [DO35]
J3  RESET  HDR_1X2  [HDR_1X2]
LED1  LED_JUMPER  [LED_JUMPER]
LED2  LED_JUMPER  [LED_JUMPER]
LED3  LED_JUMPER  [LED_JUMPER]
LED4  LED_JUMPER  [LED_JUMPER]
R1  10K  R_US  [R_204/7]
R2  100  R_US  [R_204/7]
RES15  220  RA_SIP_X4  [RN_SIP8]
RES16  220  RA_SIP_X4  [RN_SIP8]
SPARE1  SPARE18  [DIL18]
SPARE2  SPARE20  [DIL20]
SPARE3  SPARE20  [DIL20]
SPARE4  SPARE16  [DIL16]
U42  74ALS14  7414  [DIL14]

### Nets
!RSTOUS: U42.4(B:Y) ; also sheet 2
+5V: C1.1 C2.1 C3.1 C4.1 C5.1 C6.1 C7.1 C8.1 C9.1 C10.1 C11.1 C12.1 C13.1 C14.1 C15.1 C16.1 C17.1 C18.1 C19.1 C20.1 C21.1 C22.1 C25.1 C26.1 C27.1 C28.1 C29.1 C30.1 C31.1 C32.1 C33.1 C34.1 C35.1 C36.1 C37.1 C38.1 C39.1 C40.1 C41.1 C42.1 C43.1 C44.1 C45.1 C46.1 C48.1 C49.1 C50.1 C51.1 C52.1 C53.1 C54.1 C55.1 C56.1 C57.1 C58.1 C61.1 C62.1 C63.1 C64.1 C65.1 C66.1 C69.1 C70.1 C71.1 C72.1 C73.1 C74.1 C76.1 C78.1 C79.1 C80.1 CONN2.2 CONN2.4 CONN2.6 CONN2.8 CONN11.P9-4(+5V) CONN11.P9-5(+5V) CONN11.P9-6(+5V) D2.C LED1.2(A) LED2.2(A) LED3.2(A) LED4.2(A) R1.2 U5.14(P:VCC) U14.20(P:VCC) U15.20(P:VCC) U17.14(P:VCC) U18.14(P:VCC) U21.14(P:VCC) U22.14(P:VCC) U23.14(P:VCC) U30.14(P:VCC) U31.14(P:VCC) U32.14(P:VCC) U42.14(P:VCC) U45.14(P:VCC) U58.14(P:VCC) ; also sheet 1,2,3,4,5,6,7,8,10
+12V: C59.+ C68.+ CONN11.P8-3(+12V) ; also sheet 5,6,7
-12V: C60.- C67.- CONN11.P8-4(-12V) ; also sheet 5,6,7
GND: C1.2 C2.2 C3.2 C4.2 C5.2 C6.2 C7.2 C8.2 C9.2 C10.2 C11.2 C12.2 C13.2 C14.2 C15.2 C16.2 C17.2 C18.2 C19.2 C20.2 C21.2 C22.2 C25.2 C26.2 C27.2 C28.2 C29.2 C30.2 C31.2 C32.2 C33.2 C34.2 C35.2 C36.2 C37.2 C38.2 C39.2 C40.2 C41.2 C42.2 C43.2 C44.2 C45.2 C46.2 C47.- C48.2 C49.2 C50.2 C51.2 C52.2 C53.2 C54.2 C55.2 C56.2 C57.2 C58.2 C59.- C60.+ C61.2 C62.2 C63.2 C64.2 C65.2 C66.2 C67.+ C68.- C69.2 C70.2 C71.2 C72.2 C73.2 C74.2 C76.2 C78.2 C79.2 C80.2 CONN11.P8-5(GND) CONN11.P8-6(GND) CONN11.P9-1(GND) CONN11.P9-2(GND) J3.2 U5.7(P:GND) U14.10(P:GND) U15.10(P:GND) U17.7(P:GND) U18.7(P:GND) U21.7(P:GND) U22.7(P:GND) U23.7(P:GND) U30.7(P:GND) U31.7(P:GND) U32.7(P:GND) U42.7(P:GND) U45.7(P:GND) U58.7(P:GND) ; also sheet 1,2,3,4,5,6,7,8,10
PA0: RES15.8 ; also sheet 4
PA1: RES16.8 ; also sheet 4
PA2: RES15.6 ; also sheet 4
PA3: RES16.6 ; also sheet 4
PA4: RES15.4 ; also sheet 4
PA5: RES16.4 ; also sheet 4
PA6: RES15.2 ; also sheet 4
PA7: RES16.2 ; also sheet 4
RST_JFILT: C47.+ D2.A R1.1 R2.2 U42.1(A:A)
RST_JIN: J3.1 R2.1
RSTO: U42.2(A:Y) U42.3(B:A) ; also sheet 5,6,7
STS0: LED1.1(C) RES15.7
STS1: LED2.1(C) RES16.7
STS2: LED3.1(C) RES15.5
STS3: LED4.1(C) RES16.5
STS4: CONN2.7 RES15.3
STS5: CONN2.5 RES16.3
STS6: CONN2.3 RES15.1
STS7: CONN2.1 RES16.1
Unconnected: CONN11.P8-1(PGOOD) CONN11.P8-2(-5V) CONN11.P9-3(-5V) SPARE1.1 SPARE1.2 SPARE1.3 SPARE1.4 SPARE1.5 SPARE1.6 SPARE1.7 SPARE1.8 SPARE1.9 SPARE1.10 SPARE1.11 SPARE1.12 SPARE1.13 SPARE1.14 SPARE1.15 SPARE1.16 SPARE1.17 SPARE1.18 SPARE2.1 SPARE2.2 SPARE2.3 SPARE2.4 SPARE2.5 SPARE2.6 SPARE2.7 SPARE2.8 SPARE2.9 SPARE2.10 SPARE2.11 SPARE2.12 SPARE2.13 SPARE2.14 SPARE2.15 SPARE2.16 SPARE2.17 SPARE2.18 SPARE2.19 SPARE2.20 SPARE3.1 SPARE3.2 SPARE3.3 SPARE3.4 SPARE3.5 SPARE3.6 SPARE3.7 SPARE3.8 SPARE3.9 SPARE3.10 SPARE3.11 SPARE3.12 SPARE3.13 SPARE3.14 SPARE3.15 SPARE3.16 SPARE3.17 SPARE3.18 SPARE3.19 SPARE3.20 SPARE4.1 SPARE4.2 SPARE4.3 SPARE4.4 SPARE4.5 SPARE4.6 SPARE4.7 SPARE4.8 SPARE4.9 SPARE4.10 SPARE4.11 SPARE4.12 SPARE4.13 SPARE4.14 SPARE4.15 SPARE4.16 U15.7(C:A) U15.8(C:B) U15.9(C:Y) U21.1(A:A) U21.2(A:Y) U21.3(B:A) U21.4(B:Y) U21.5(C:A) U21.6(C:Y) U21.12(F:Y) U21.13(F:A) U31.8(B:!Q) U31.9(B:Q) U31.10(B:!PRE) U31.11(B:CLK) U31.12(B:D) U31.13(B:!CLR) U42.5(C:A) U42.6(C:Y) U42.8(D:Y) U42.9(D:A) U42.10(E:Y) U42.11(E:A) U42.12(F:Y) U42.13(F:A) U58.1(A:A) U58.2(A:B) U58.3(A:Y) U58.11(D:Y) U58.12(D:A) U58.13(D:B)

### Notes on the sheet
- Optional External
  Reset Switch
- (c) 1988,89 George Scolaro
  941 Chehalis Dr.
  Sunnyvale  CA, 94087
- 532 Baby AT
- By-pass & Connectors
- retrotronics.org | n/a | 1D+

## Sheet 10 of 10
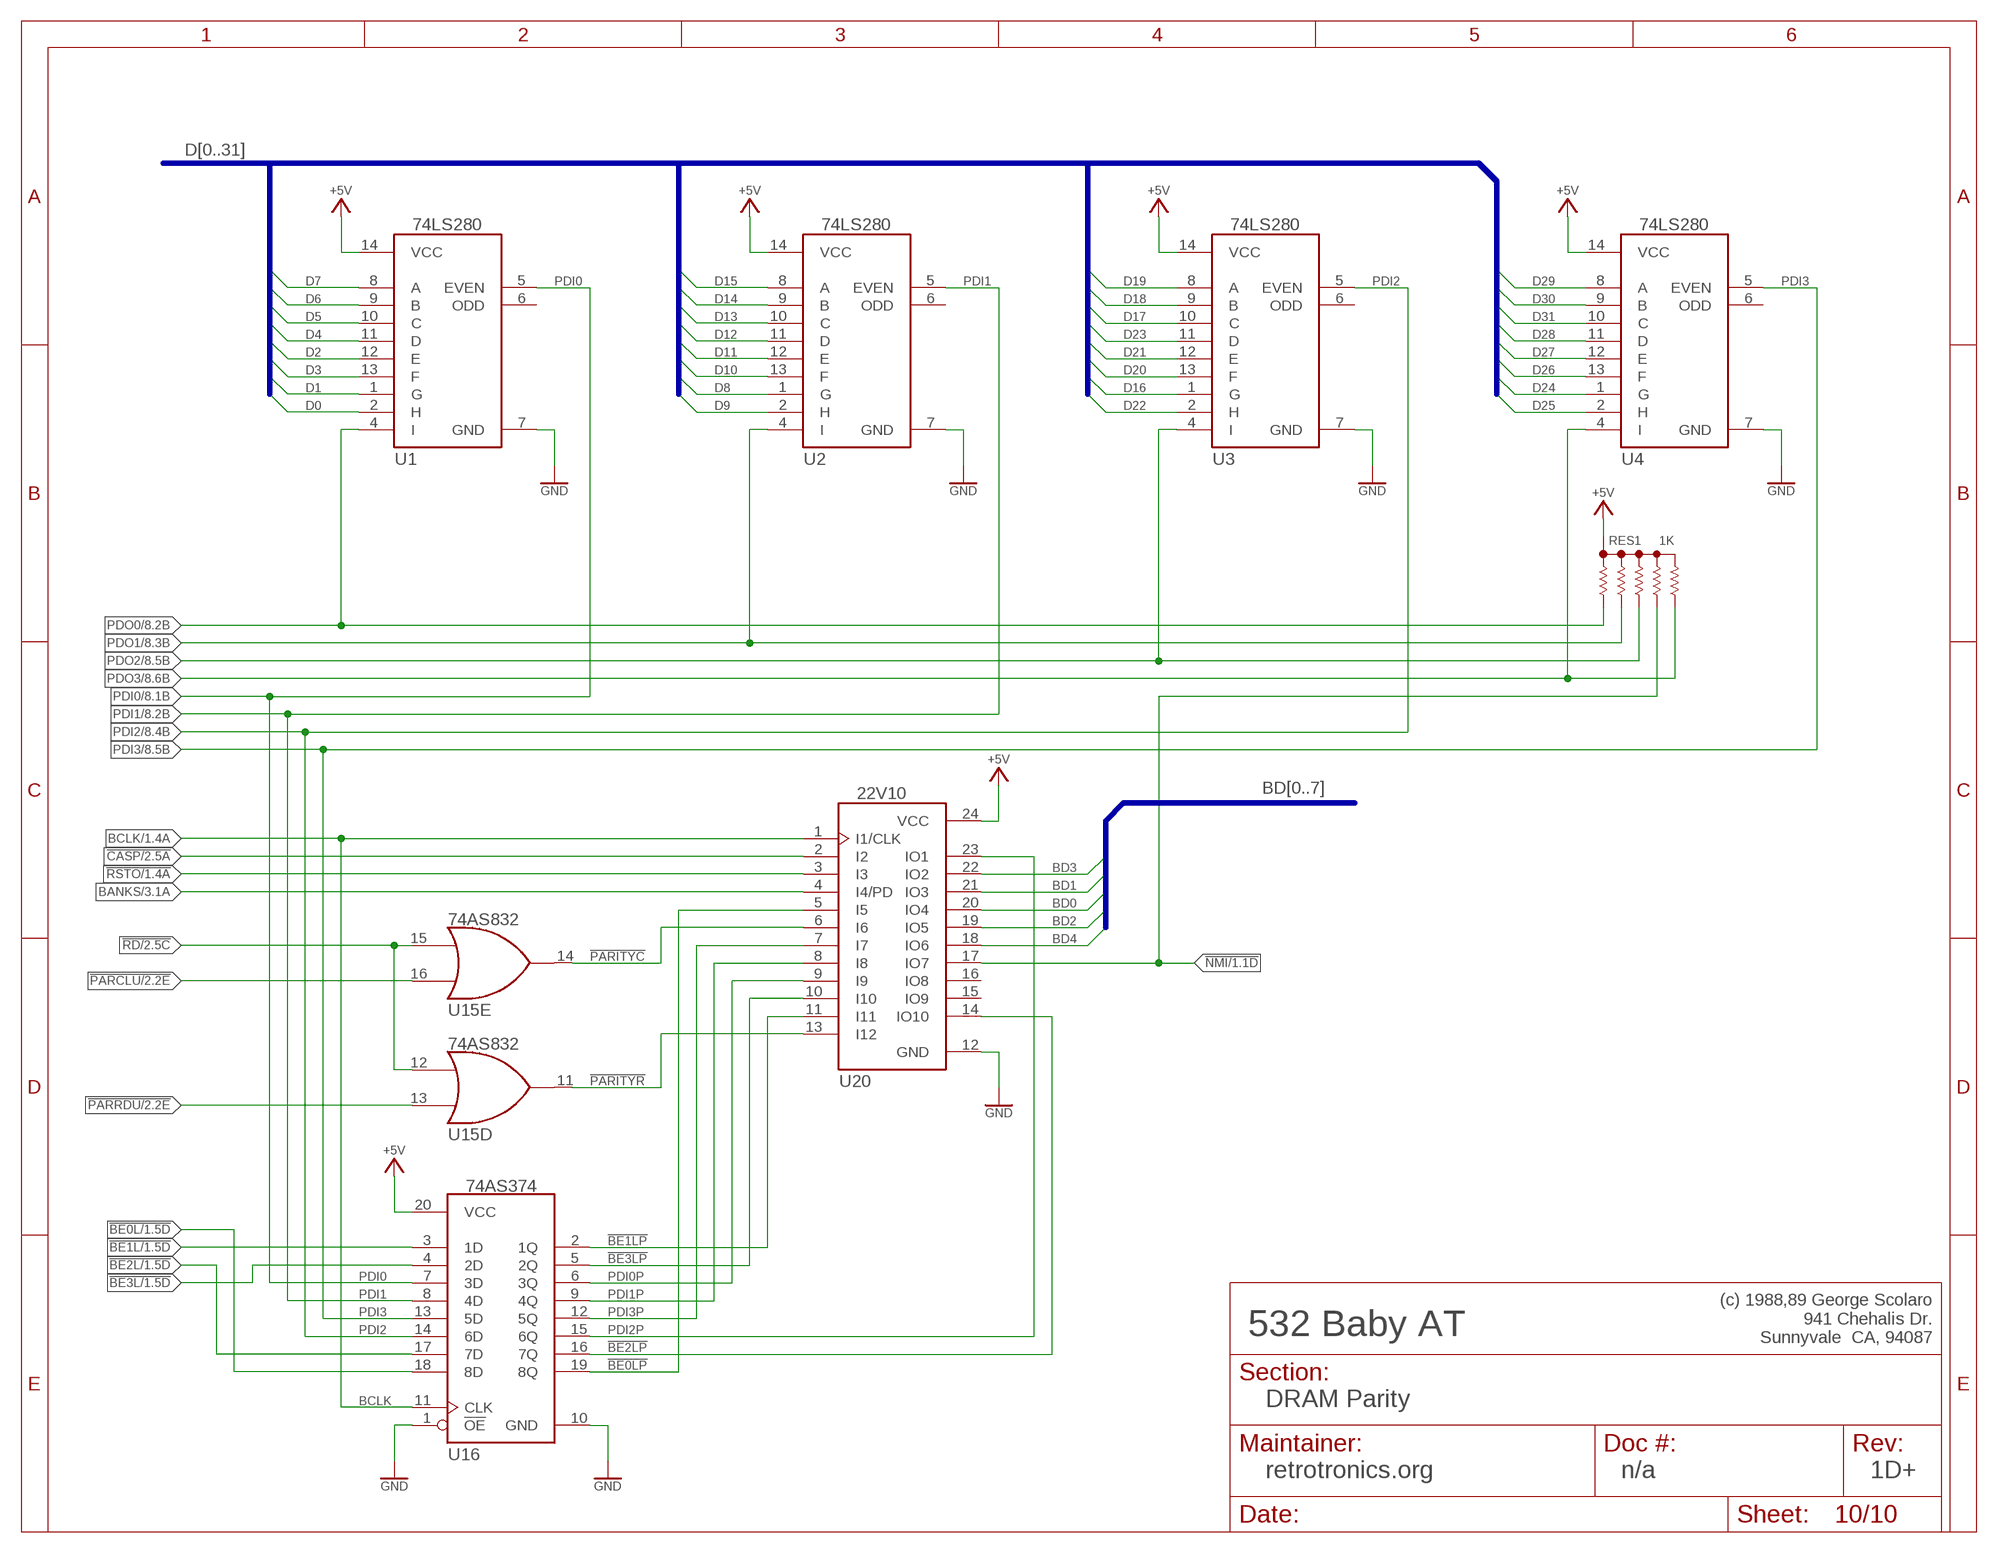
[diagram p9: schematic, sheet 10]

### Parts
RES1  1K  RNET_X5  [RN_SIP6]
U1  74LS280  74280  [DIL14]
U2  74LS280  74280  [DIL14]
U3  74LS280  74280  [DIL14]
U4  74LS280  74280  [DIL14]
U16  74AS374  74374  [DIL20_ROUND]
U20  22V10  22V10P  [DIL24]

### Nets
!BE0L: U16.18(8D) ; also sheet 1,3
!BE0LP: U16.19(8Q) U20.5(I5)
!BE1L: U16.3(1D) ; also sheet 1,3
!BE1LP: U16.2(1Q) U20.11(I11)
!BE2L: U16.17(7D) ; also sheet 1,3
!BE2LP: U16.16(7Q) U20.14(IO10)
!BE3L: U16.4(2D) ; also sheet 1,3
!BE3LP: U16.5(2Q) U20.10(I10)
!CASP: U20.2(I2) ; also sheet 2
!NMI: RES1.5 U20.17(IO7) ; also sheet 1
!PARCLU: U15.16(E:B) ; also sheet 2
!PARITYC: U15.14(E:Y) U20.6(I6)
!PARITYR: U15.11(D:Y) U20.13(I12)
!PARRDU: U15.13(D:B) ; also sheet 2
!RD: U15.12(D:A) U15.15(E:A) ; also sheet 2,4,5,6,7
!RSTO: U20.3(I3) ; also sheet 1,2,4,5
+5V: RES1.1 U1.14(VCC) U2.14(VCC) U3.14(VCC) U4.14(VCC) U16.20(VCC) U20.24(VCC) ; also sheet 1,2,3,4,5,6,7,8,9
BANKS: U20.4(I4/PD) ; also sheet 3
BCLK: U16.11(CLK) U20.1(I1/CLK) ; also sheet 1,2
BD0: U20.20(IO4) ; also sheet 2,4,5,6,7
BD1: U20.21(IO3) ; also sheet 2,4,5,6,7
BD2: U20.19(IO5) ; also sheet 2,4,5,6,7
BD3: U20.22(IO2) ; also sheet 2,4,5,6,7
BD4: U20.18(IO6) ; also sheet 2,4,5,6,7
D0: U1.2(H) ; also sheet 1,4,8
D1: U1.1(G) ; also sheet 1,4,8
D2: U1.12(E) ; also sheet 1,4,8
D3: U1.13(F) ; also sheet 1,4,8
D4: U1.11(D) ; also sheet 1,4,8
D5: U1.10(C) ; also sheet 1,4,8
D6: U1.9(B) ; also sheet 1,4,8
D7: U1.8(A) ; also sheet 1,4,8
D8: U2.1(G) ; also sheet 1,8
D9: U2.2(H) ; also sheet 1,8
D10: U2.13(F) ; also sheet 1,8
D11: U2.12(E) ; also sheet 1,8
D12: U2.11(D) ; also sheet 1,8
D13: U2.10(C) ; also sheet 1,8
D14: U2.9(B) ; also sheet 1,8
D15: U2.8(A) ; also sheet 1,8
D16: U3.1(G) ; also sheet 1,8
D17: U3.10(C) ; also sheet 1,8
D18: U3.9(B) ; also sheet 1,8
D19: U3.8(A) ; also sheet 1,8
D20: U3.13(F) ; also sheet 1,8
D21: U3.12(E) ; also sheet 1,8
D22: U3.2(H) ; also sheet 1,8
D23: U3.11(D) ; also sheet 1,8
D24: U4.1(G) ; also sheet 1,8
D25: U4.2(H) ; also sheet 1,8
D26: U4.13(F) ; also sheet 1,8
D27: U4.12(E) ; also sheet 1,8
D28: U4.11(D) ; also sheet 1,8
D29: U4.8(A) ; also sheet 1,8
D30: U4.9(B) ; also sheet 1,8
D31: U4.10(C) ; also sheet 1,8
GND: U1.7(GND) U2.7(GND) U3.7(GND) U4.7(GND) U16.1(!OE) U16.10(GND) U20.12(GND) ; also sheet 1,2,3,4,5,6,7,8,9
PDI0: U1.5(EVEN) U16.7(3D) ; also sheet 8
PDI0P: U16.6(3Q) U20.9(I9)
PDI1: U2.5(EVEN) U16.8(4D) ; also sheet 8
PDI1P: U16.9(4Q) U20.8(I8)
PDI2: U3.5(EVEN) U16.14(6D) ; also sheet 8
PDI2P: U16.15(6Q) U20.23(IO1)
PDI3: U4.5(EVEN) U16.13(5D) ; also sheet 8
PDI3P: U16.12(5Q) U20.7(I7)
PDO0: RES1.2 U1.4(I) ; also sheet 8
PDO1: RES1.3 U2.4(I) ; also sheet 8
PDO2: RES1.4 U3.4(I) ; also sheet 8
PDO3: RES1.6 U4.4(I) ; also sheet 8
Unconnected: U1.6(ODD) U2.6(ODD) U3.6(ODD) U4.6(ODD) U20.15(IO9) U20.16(IO8)

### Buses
D[0..31]
BD[0..7]

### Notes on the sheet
- (c) 1988,89 George Scolaro
  941 Chehalis Dr.
  Sunnyvale  CA, 94087
- 532 Baby AT
- DRAM Parity
- retrotronics.org | n/a | 1D+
